(* Logix 5000 AddOnInstructionDefinition export Banner_Q90R2_KD_Param_v4; software revision 33.00 *)

TYPE Banner_IOL_Port_v4 :   // UDT that has all of the data items necessary to communicate with a specific Port on a IO-Link Master
STRUCT
   Port_Controlled : INT;   // Each bit represents a port on an IO-Link Master. Set to 1 to tell AOI to control that port.
   Port_Activate : INT;   // Each bit represents a port on an IO-Link Master. When ON that port will process any commands in queue.
   Port_Read : INT;   // Each bit represents a port on an IO-Link Master. Used to determine when device AOI has requested a Read command.
   Port_Write : INT;   // Each bit represents a port on an IO-Link Master. Used to determine when device AOI has requested a Write command.
   Port_RW_Complete : INT;   // Each bit represents a port on an IO-Link Master. Tells device AOI that Read or Write request has been completed.
   Port_Device_Read : INT;
   Data_Transfer : SINT[190];   // Array to transfer data from IO-Master to device AOIs.
END_STRUCT
END_TYPE

TYPE Banner_Q90R2KD_Config_v4 :
STRUCT
   Response_Speed : SINT;   // 0 = Fast, 1 = Medium, 2 = Slow
   Detection_Sensitivity : SINT;   // 0 = High, 1 = Standard.
   LEDs_Disabled : SINT;   // 0 = Enabled, 1 = Disabled.
   Output_Polarity : SINT;   // 0 = NPN, 1 = PNP
   Process_Data_Measurement : SINT;   // 0 = Radial, 1 = Rectangular.
   Remote_Input_Mode : SINT;   // 0 = Disabled, 1 = Teach
   Amplitude_Threshold : DINT;   // 100 to 100000. Minimum amplitude required for target detection.
   Limit_Filter_Enabled : SINT;   // 0 = Disabled, 1 = Enabled. Rate of change filter for the distance meansurement.
   Limit_Filter_Positive_Hold_Time : DINT;   // 50 to 3600000. Hold time for when distance change exceeds positive window.
   Limit_Filter_Negative_Hold_Time : DINT;   // 50 to 3600000. Hold time for when distance change exceeds negative window.
   Limit_Filter_Positive_Distance : DINT;   // 0 to 1000. Window size for distance changes going away from sensor (set 0 to disable)
   Limit_Filter_Negative_Distance : DINT;   // 0 to 1000. Window size for distance changes going towards sensor (set 0 to disable)
   Primary_Output_Mode : SINT;   // 0 = Independent Output, 1 = Complementary Output, 2 = Pulse Frequency Output.
   Secondary_Output_Mode : SINT;   // 0 = Independent Output, 1 = Complementary Output, 2 = Pulse Frequency Output.
END_STRUCT
END_TYPE

TYPE Banner_Q90R2KD_Direct_v4 :
STRUCT
   Master_Cycle_Time : INT;
   Min_Cycle_Time : INT;
   M_Sequence_Capability : INT;
   IO_Link_Version_ID : INT;
   Process_Data_Input_Length : INT;
   Process_Data_Output_Length : INT;
   Combined_Vendor_ID : DINT;   // IO-Link Vendor ID
   Vendor_ID1 : INT;
   Vendor_ID2 : INT;
   Combined_Device_ID : DINT;   // IO-Link Device ID
   Device_ID1 : INT;
   Device_ID2 : INT;
   Device_ID3 : INT;
END_STRUCT
END_TYPE

TYPE Banner_Q90R2KD_Pulse_v4 :
STRUCT
   Measurement : SINT;   // 0 = Distance or Y, 1 = Velocity. Measurement to use for PFM output.
   Frequency_SP1 : INT;   // 100 to 600. The frequency corresponding to a target at the SP1 measurement.
   Frequency_SP2 : INT;   // 100 to 600. The frequency corresponding to a target at the SP1 measurement.
   Loss_of_Signal : SINT;   // 0 = Hold, 1 = Low, 2 = High.
   Distance_SP1 : DINT;   // Distance SP1 swithc point in Switch or Window mode.
   Distance_SP2 : DINT;   // Distance SP2 switch point in Window mode only.
   Y_SP1 : DINT;   // Y SP1 switch point in Switch or Window mode.
   Y_SP2 : DINT;   // Y SP2 switch point in Window mode only.
   Velocity_SP1 : DINT;   // Velocity SP1 switch point.
   Velocity_SP2 : DINT;   // Velocity SP2 switch point.
END_STRUCT
END_TYPE

TYPE Banner_Q90R2KD_RD_v4 :   // UDT that stores the Read Data for a Q90R2KD.
STRUCT
   Direct : Banner_Q90R2KD_Direct_v4;   // Direct Parameters.
   Serial_Number : STRING;
   Teach_Status : Banner_Q90R2KD_Teach_Status_v4;
   Status : Banner_Q90R2KD_Status_v4;
   All_Time_Run_Time : DINT;   // Read only counter that tracks the total time sensor has been running since manufacture. Value in Hours.
END_STRUCT
END_TYPE

TYPE Banner_Q90R2KD_SSC_v4 :
STRUCT
   Distance_SP1 : DINT;   // SP1 switch point in Switch or Window mode.
   Distance_SP2 : DINT;   // SP2 switch point in Window mode only.
   Distance_Hysteresis : INT;
   Y_SP1 : DINT;   // Y SP1 siwtch point in Switch or Window mode.
   Y_SP2 : DINT;   // Y SP2 switch point in Window mode only.
   Y_Hysteresis : DINT;
   Switch_Point_Logic : INT;   // 0 = Light Operate - Output is On while target is detected, 1 = Dark Operate - Output is Off while target is detected.
   Distance_Y_Setpoint_Mode : INT;   // 1 = Switch Mode/Single Point Mode, 2 = Window Mode.
   Delay_On : DINT;   // 0 to 60000.
   Delay_Off : DINT;   // 0 to 60000.
   Distance_Window_Size : DINT;   // This will set the size of the distance window after a teach. Window size will be +/- xmm where x is the value written.
   Distance_User_Teach_Offset : DINT;   // Distance offset applied to taught switch point.
   Beam_Angle_Window_Size : DINT;   // This will set the size of the beam angle window after a teach. Window size will be +/- xmm where x is the value written.
   Beam_Angle_User_Teach_Offset : DINT;   // Beam Angle offset applied to taught switch point.
   X_Window_Size : DINT;   // This will set the size of the X window after a teach. Window size will be +/- xmm where x is the value written.
   X_User_Teach_Offset : DINT;   // X offset applied to taught switch point.
   Y_Window_Size : DINT;   // This will set the size of the Y window after a teach. Window size will be +/- xmm where x is the value written.
   Y_User_Teach_Offset : DINT;   // Y offset applied to taught switch point.
   Peak_Select_Mode : SINT;   // 0 = First Peak, 1 = Strongest Peak.
   Beam_Angle_SP1 : INT;   // Beam Angle SP1 Switch point.
   Beam_Angle_SP2 : INT;   // Beam Angle SP2 switch point.
   Beam_Angle_Hysteresis : SINT;   // Hysteresis value for the beam angle switchpoint.
   X_SP1 : DINT;   // X SP1 switch point.
   X_SP2 : DINT;   // X SP2 switch point.
   X_Hysteresis : INT;   // Hysteresis value for the X switchpoint.
END_STRUCT
END_TYPE

TYPE Banner_Q90R2KD_Status_v4 :
STRUCT
   SSC1_State : SINT;   // 0 = Inactive, 1 = Active.
   SSC1_Stability : SINT;   // 0 = No target, 1 = Marginal target, 2 = Strong target.
   SSC1_Distance_or_X : DINT;
   SSC1_Beam_Angle_or_Y : DINT;
   SSC1_Velocity : DINT;
   SSC1_Signal_Strength : SINT;
   SSC2_State : SINT;   // 0 = Inactive, 1 = Active.
   SSC2_Stability : SINT;   // 0 = No target, 1 = Marginal target, 2 = Strong target.
   SSC2_Distance_or_X : DINT;
   SSC2_Beam_Angle_or_Y : DINT;
   SSC2_Velocity : DINT;
   SSC2_Signal_Strength : SINT;
   Fault_Status : SINT;   // 0 = No fault present, 1 = Fault present.
   Temperature : DINT;
   Last_Temperature : DINT;
END_STRUCT
END_TYPE

TYPE Banner_Q90R2KD_Target_Filters_v4 :
STRUCT
   Detection_Area : SINT;   // 0 = Radial, 1 = Rectangular.
   Min_Active_Sensing_Distance : DINT;   // Near radial distance measurement limit of sensing range.
   Max_Active_Sensing_Distance : DINT;   // Far radial distance measurement limit of sensing range.
   Min_Active_Sensing_Y : DINT;   // Near Y coordinate measurement limit of sensing range.
   Max_Active_Sensing_Y : DINT;   // Far Y coordinate measurment limit of sensing range.
   Velocity_Filter : INT;   // 0 = All Target Velocities, 1 = Dynamix Targets Only, 2 = Approaching Targets Only, 3 = Receding Targets Only, 4 = Custom.
   Min_Velocity : DINT;   // Minimum velocity limit of sensing range.
   Max_Velocity : DINT;   // Maximum velocity lmiit of sensing range.
   Velocity_Hysteresis : DINT;   // Hysteresis value for the velocity switchpoint.
END_STRUCT
END_TYPE

TYPE Banner_Q90R2KD_Teach_Status_v4 :
STRUCT
   Teach_State : SINT;   // 0 = Idle, 1 = SP1 Success, 2 = SP2 Success, 3 = SP1 SP2 Success, 4 = Wait for command, 5 = Busy, 7 = Error
   SP1_TP1 : SINT;
   SP1_TP2 : SINT;
   SP2_TP1 : SINT;
   SP2_TP2 : SINT;
END_STRUCT
END_TYPE

TYPE Banner_Q90R2KD_v4 :   // All of the parameters for a Q90R2KD.
STRUCT
   Initial_Global_Read : BOOL;   // Determines if all of the IO-Link data has been read into the PLC yet
   Command : INT;   // Value placed in here will activate a read or write to a specifc IO-Link Index
   Read : Banner_Q90R2KD_RD_v4;   // Read Only Data
   Write : Banner_Q90R2KD_WD_v4;   // Write Data
   Reset : BOOL;   // Resets AOI. This will force a complete parameter read of the sensor.
END_STRUCT
END_TYPE

TYPE Banner_Q90R2KD_WD_v4 :   // UDT that stores the Write Data for a Q90R2KD.
STRUCT
   System_Command : INT;   // See IODD file for list of commands that can be activated via the System Command interface
   Teach_in_Channel : SINT;   // 0 = Default, 1 = BDC1, 2 = BDC2
   SSC1 : Banner_Q90R2KD_SSC_v4;
   SSC2 : Banner_Q90R2KD_SSC_v4;
   Config : Banner_Q90R2KD_Config_v4;
   Resettable_Run_Time : DINT;
   All_Time_Run_Time_Event_Time : DINT;
   Resettable_Run_Time_Event_Time : DINT;
   Target_Filters : Banner_Q90R2KD_Target_Filters_v4;
   Pulse1 : Banner_Q90R2KD_Pulse_v4;
   Pulse2 : Banner_Q90R2KD_Pulse_v4;
END_STRUCT
END_TYPE

ADD_ON_INSTRUCTION Banner_Q90R2_KD_Param_v4   (* revision 4.0, vendor Banner Engineering *)
// AOI to read and write parameter data to an IO-Link Q90R2 Dual Discrete.
VAR_IN_OUT
   Q90R2KD : Banner_Q90R2KD_v4; {required}
   Port_Data : Banner_IOL_Port_v4; {required}
END_VAR
VAR_INPUT
   Port : DINT; {required}
END_VAR
VAR
   Local_Control : DINT; {access None}
   Global_Read_Command_Value : INT; {access None}
   Global_Write_Command_Value : INT; {access None}
   Command_Being_Processed : BOOL; {access None}
   Update_Archive : BOOL; {access None}
   Index_Write_Inprocess : DINT; {access None}
   Index_Write_Control : DINT; {access None}
   Inprocess_Index : DINT; {access None}
END_VAR

ROUTINE Logic   (* ladder *)
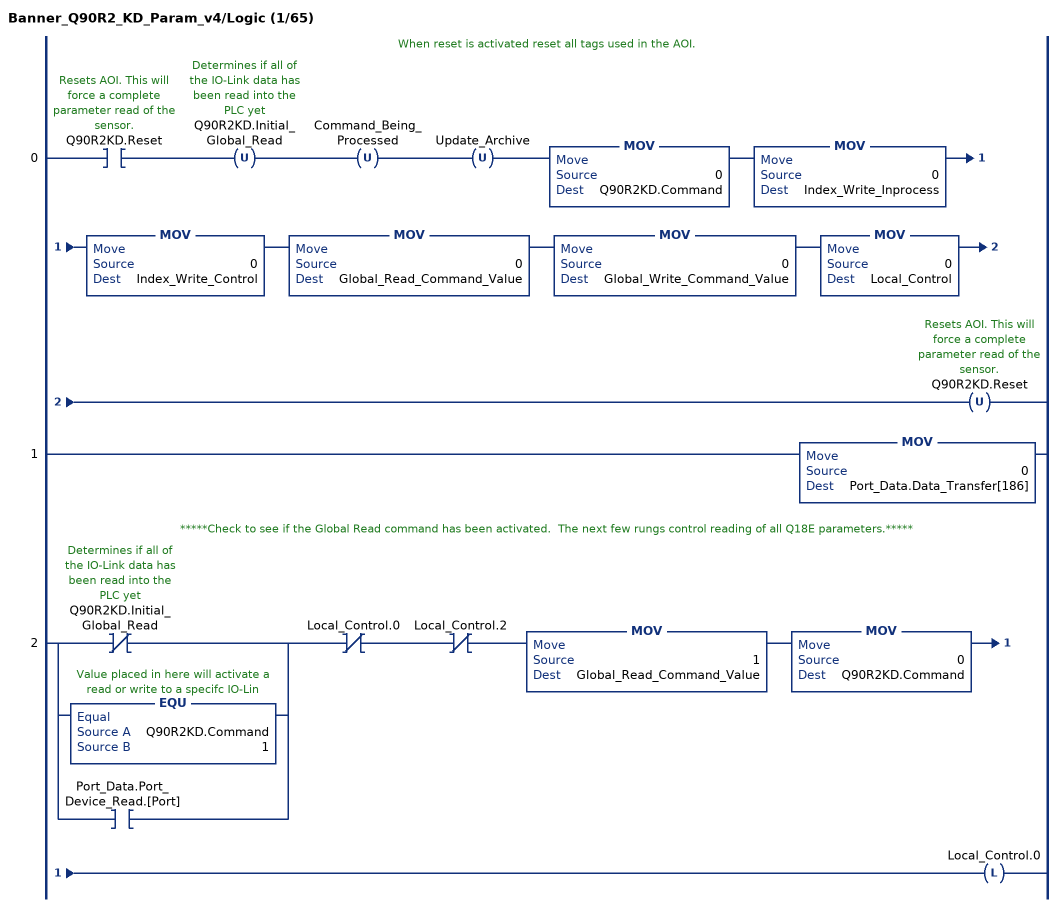
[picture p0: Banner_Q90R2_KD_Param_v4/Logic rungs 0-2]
   // When reset is activated reset all tags used in the AOI.
   0: XIC(Q90R2KD.Reset)OTU(Q90R2KD.Initial_Global_Read)OTU(Command_Being_Processed)OTU(Update_Archive)MOV(0,Q90R2KD.Command)MOV(0,Index_Write_Inprocess)MOV(0,Index_Write_Control)MOV(0,Global_Read_Command_Value)MOV(0,Global_Write_Command_Value)MOV(0,Local_Control)OTU(Q90R2KD.Reset);
   1: MOV(0,Port_Data.Data_Transfer[186]);
   // *****Check to see if the Global Read command has been activated.  The next few rungs control reading of all Q18E parameters.*****
   2: [XIO(Q90R2KD.Initial_Global_Read) ,EQU(Q90R2KD.Command,1) ,XIC(Port_Data.Port_Device_Read.[Port]) ]XIO(Local_Control.0)XIO(Local_Control.2)MOV(1,Global_Read_Command_Value)MOV(0,Q90R2KD.Command)OTL(Local_Control.0);
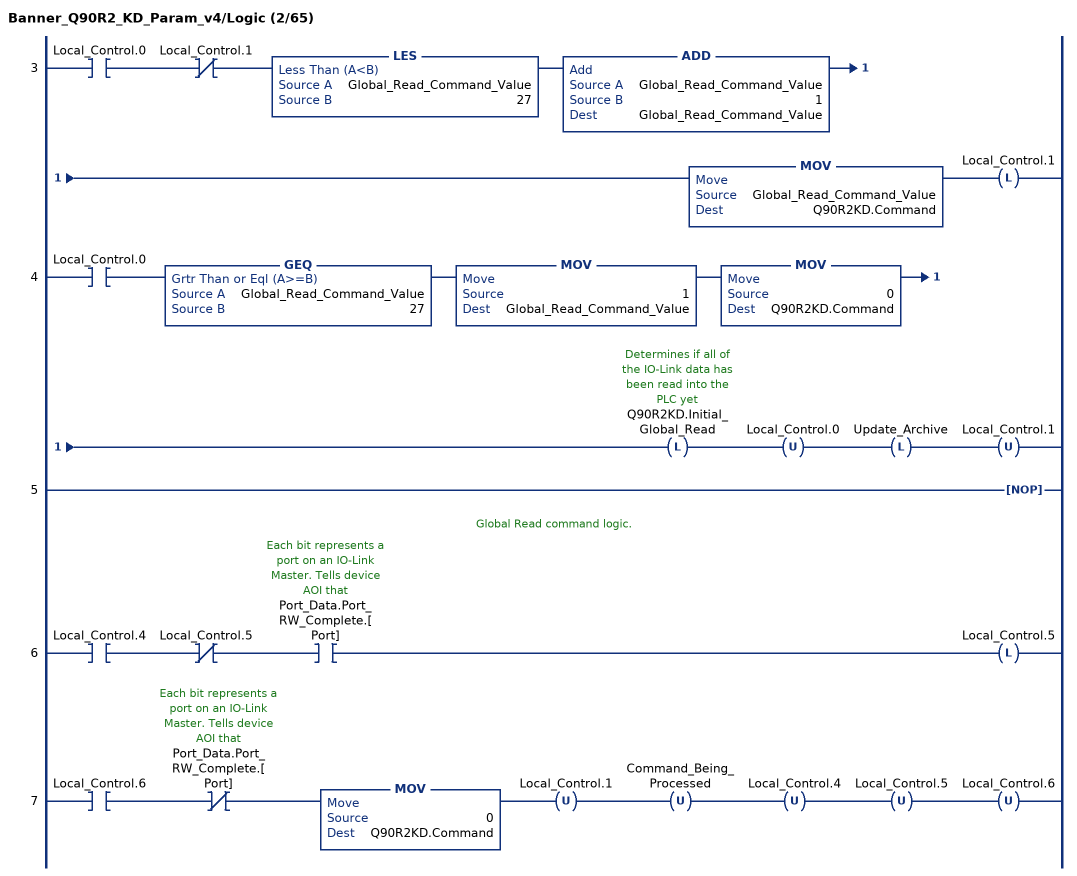
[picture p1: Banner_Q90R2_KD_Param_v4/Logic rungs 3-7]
   3: XIC(Local_Control.0)XIO(Local_Control.1)LES(Global_Read_Command_Value,27)ADD(Global_Read_Command_Value,1,Global_Read_Command_Value)MOV(Global_Read_Command_Value,Q90R2KD.Command)OTL(Local_Control.1);
   4: XIC(Local_Control.0)GEQ(Global_Read_Command_Value,27)MOV(1,Global_Read_Command_Value)MOV(0,Q90R2KD.Command)OTL(Q90R2KD.Initial_Global_Read)OTU(Local_Control.0)OTL(Update_Archive)OTU(Local_Control.1);
   5: NOP();
   // Global Read command logic.
   6: XIC(Local_Control.4)XIO(Local_Control.5)XIC(Port_Data.Port_RW_Complete.[Port])OTL(Local_Control.5);
   7: XIC(Local_Control.6)XIO(Port_Data.Port_RW_Complete.[Port])MOV(0,Q90R2KD.Command)OTU(Local_Control.1)OTU(Command_Being_Processed)OTU(Local_Control.4)OTU(Local_Control.5)OTU(Local_Control.6);
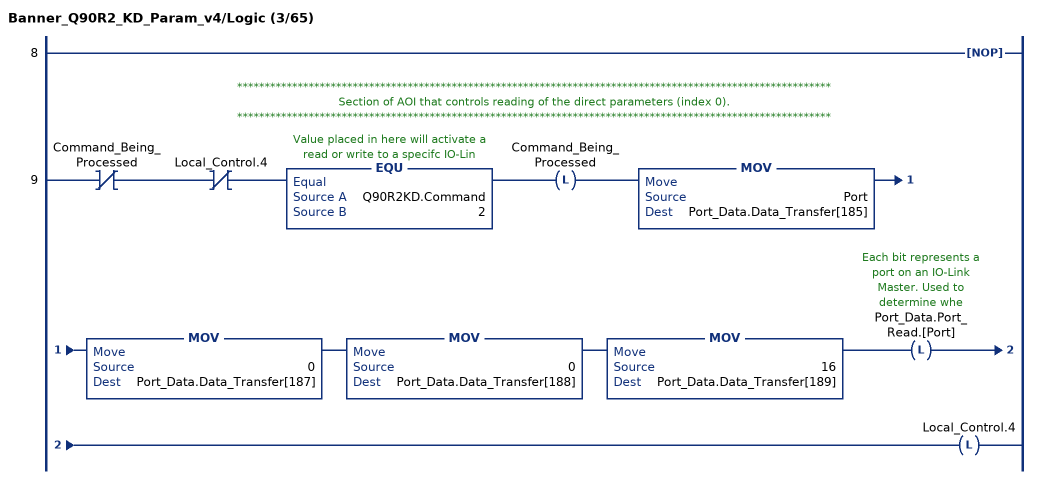
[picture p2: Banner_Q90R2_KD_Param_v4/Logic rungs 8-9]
   8: NOP();
   // ************************************************************************************************************
   // Section of AOI that controls reading of the direct parameters (index 0).
   // ************************************************************************************************************
   9: XIO(Command_Being_Processed)XIO(Local_Control.4)EQU(Q90R2KD.Command,2)OTL(Command_Being_Processed)MOV(Port,Port_Data.Data_Transfer[185])MOV(0,Port_Data.Data_Transfer[187])MOV(0,Port_Data.Data_Transfer[188])MOV(16,Port_Data.Data_Transfer[189])OTL(Port_Data.Port_Read.[Port])OTL(Local_Control.4);
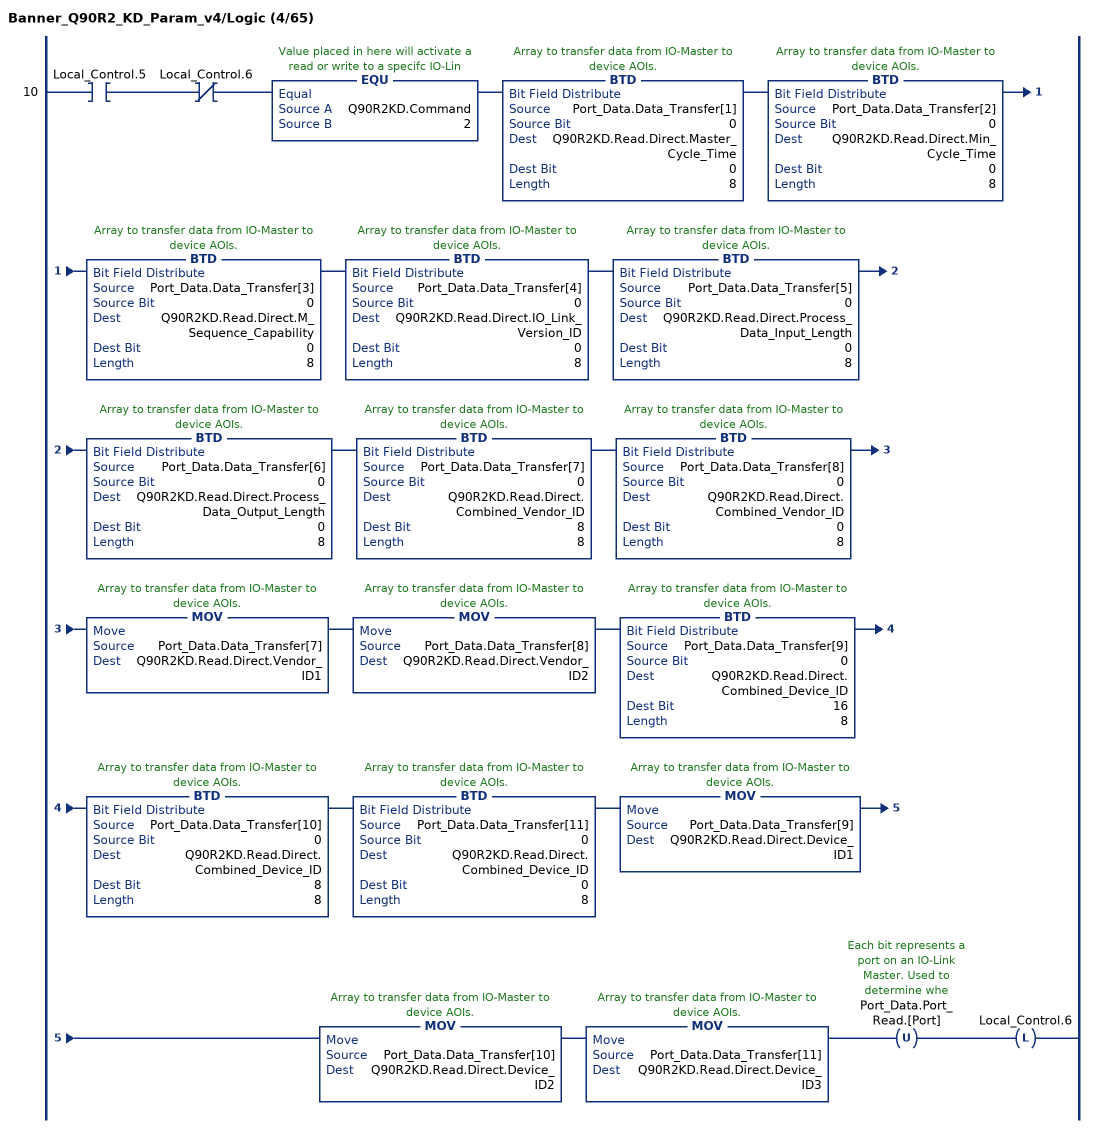
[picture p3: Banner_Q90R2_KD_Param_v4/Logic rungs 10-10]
   10: XIC(Local_Control.5)XIO(Local_Control.6)EQU(Q90R2KD.Command,2)BTD(Port_Data.Data_Transfer[1],0,Q90R2KD.Read.Direct.Master_Cycle_Time,0,8)BTD(Port_Data.Data_Transfer[2],0,Q90R2KD.Read.Direct.Min_Cycle_Time,0,8)BTD(Port_Data.Data_Transfer[3],0,Q90R2KD.Read.Direct.M_Sequence_Capability,0,8)BTD(Port_Data.Data_Transfer[4],0,Q90R2KD.Read.Direct.IO_Link_Version_ID,0,8)BTD(Port_Data.Data_Transfer[5],0,Q90R2KD.Read.Direct.Process_Data_Input_Length,0,8)BTD(Port_Data.Data_Transfer[6],0,Q90R2KD.Read.Direct.Process_Data_Output_Length,0,8)BTD(Port_Data.Data_Transfer[7],0,Q90R2KD.Read.Direct.Combined_Vendor_ID,8,8)BTD(Port_Data.Data_Transfer[8],0,Q90R2KD.Read.Direct.Combined_Vendor_ID,0,8)MOV(Port_Data.Data_Transfer[7],Q90R2KD.Read.Direct.Vendor_ID1)MOV(Port_Data.Data_Transfer[8],Q90R2KD.Read.Direct.Vendor_ID2)BTD(Port_Data.Data_Transfer[9],0,Q90R2KD.Read.Direct.Combined_Device_ID,16,8)BTD(Port_Data.Data_Transfer[10],0,Q90R2KD.Read.Direct.Combined_Device_ID,8,8)BTD(Port_Data.Data_Transfer[11],0,Q90R2KD.Read.Direct.Combined_Device_ID,0,8)MOV(Port_Data.Data_Transfer[9],Q90R2KD.Read.Direct.Device_ID1)MOV(Port_Data.Data_Transfer[10],Q90R2KD.Read.Direct.Device_ID2)MOV(Port_Data.Data_Transfer[11],Q90R2KD.Read.Direct.Device_ID3)OTU(Port_Data.Port_Read.[Port])OTL(Local_Control.6);
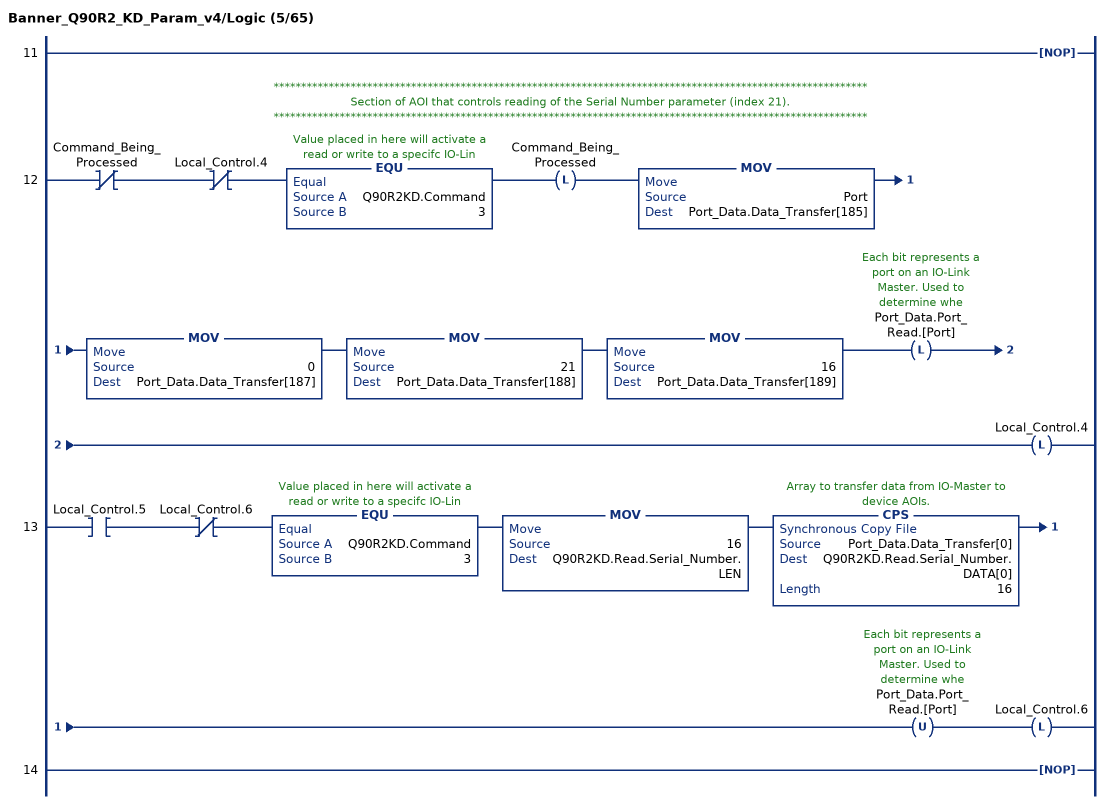
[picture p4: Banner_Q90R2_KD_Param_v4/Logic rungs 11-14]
   11: NOP();
   // ************************************************************************************************************
   // Section of AOI that controls reading of the Serial Number parameter (index 21).
   // ************************************************************************************************************
   12: XIO(Command_Being_Processed)XIO(Local_Control.4)EQU(Q90R2KD.Command,3)OTL(Command_Being_Processed)MOV(Port,Port_Data.Data_Transfer[185])MOV(0,Port_Data.Data_Transfer[187])MOV(21,Port_Data.Data_Transfer[188])MOV(16,Port_Data.Data_Transfer[189])OTL(Port_Data.Port_Read.[Port])OTL(Local_Control.4);
   13: XIC(Local_Control.5)XIO(Local_Control.6)EQU(Q90R2KD.Command,3)MOV(16,Q90R2KD.Read.Serial_Number.LEN)CPS(Port_Data.Data_Transfer[0],Q90R2KD.Read.Serial_Number.DATA[0],16)OTU(Port_Data.Port_Read.[Port])OTL(Local_Control.6);
   14: NOP();
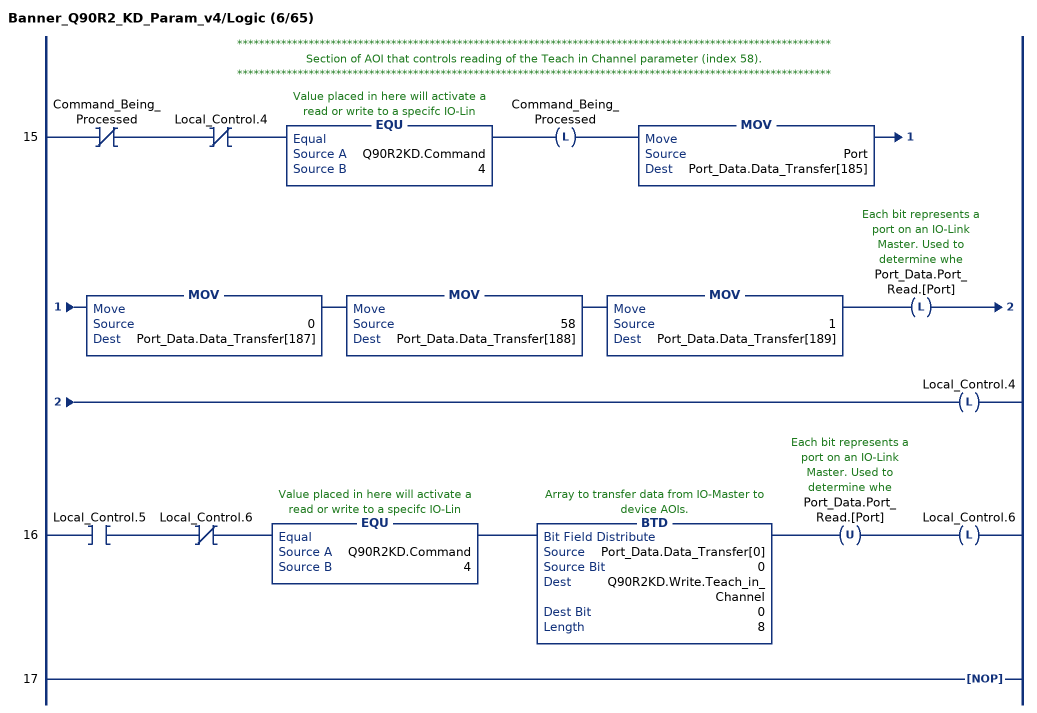
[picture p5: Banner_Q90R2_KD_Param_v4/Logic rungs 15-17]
   // ************************************************************************************************************
   // Section of AOI that controls reading of the Teach in Channel parameter (index 58).
   // ************************************************************************************************************
   15: XIO(Command_Being_Processed)XIO(Local_Control.4)EQU(Q90R2KD.Command,4)OTL(Command_Being_Processed)MOV(Port,Port_Data.Data_Transfer[185])MOV(0,Port_Data.Data_Transfer[187])MOV(58,Port_Data.Data_Transfer[188])MOV(1,Port_Data.Data_Transfer[189])OTL(Port_Data.Port_Read.[Port])OTL(Local_Control.4);
   16: XIC(Local_Control.5)XIO(Local_Control.6)EQU(Q90R2KD.Command,4)BTD(Port_Data.Data_Transfer[0],0,Q90R2KD.Write.Teach_in_Channel,0,8)OTU(Port_Data.Port_Read.[Port])OTL(Local_Control.6);
   17: NOP();
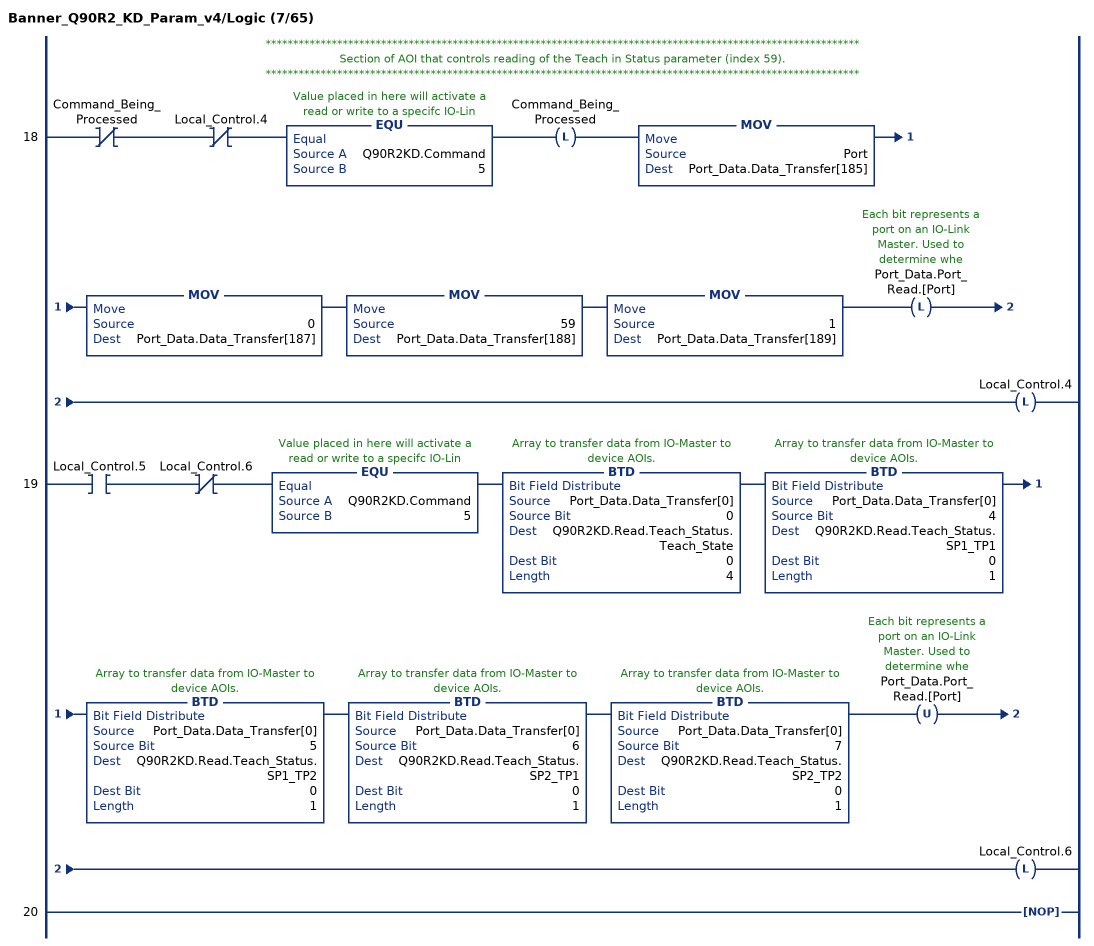
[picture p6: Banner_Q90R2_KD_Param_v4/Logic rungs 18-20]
   // ************************************************************************************************************
   // Section of AOI that controls reading of the Teach in Status parameter (index 59).
   // ************************************************************************************************************
   18: XIO(Command_Being_Processed)XIO(Local_Control.4)EQU(Q90R2KD.Command,5)OTL(Command_Being_Processed)MOV(Port,Port_Data.Data_Transfer[185])MOV(0,Port_Data.Data_Transfer[187])MOV(59,Port_Data.Data_Transfer[188])MOV(1,Port_Data.Data_Transfer[189])OTL(Port_Data.Port_Read.[Port])OTL(Local_Control.4);
   19: XIC(Local_Control.5)XIO(Local_Control.6)EQU(Q90R2KD.Command,5)BTD(Port_Data.Data_Transfer[0],0,Q90R2KD.Read.Teach_Status.Teach_State,0,4)BTD(Port_Data.Data_Transfer[0],4,Q90R2KD.Read.Teach_Status.SP1_TP1,0,1)BTD(Port_Data.Data_Transfer[0],5,Q90R2KD.Read.Teach_Status.SP1_TP2,0,1)BTD(Port_Data.Data_Transfer[0],6,Q90R2KD.Read.Teach_Status.SP2_TP1,0,1)BTD(Port_Data.Data_Transfer[0],7,Q90R2KD.Read.Teach_Status.SP2_TP2,0,1)OTU(Port_Data.Port_Read.[Port])OTL(Local_Control.6);
   20: NOP();
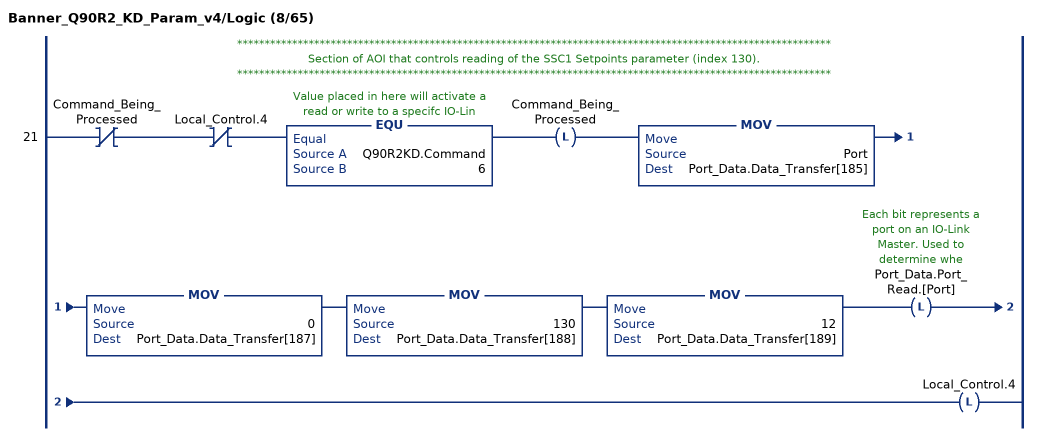
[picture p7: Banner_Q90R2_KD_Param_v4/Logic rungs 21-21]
   // ************************************************************************************************************
   // Section of AOI that controls reading of the SSC1 Setpoints parameter (index 130).
   // ************************************************************************************************************
   21: XIO(Command_Being_Processed)XIO(Local_Control.4)EQU(Q90R2KD.Command,6)OTL(Command_Being_Processed)MOV(Port,Port_Data.Data_Transfer[185])MOV(0,Port_Data.Data_Transfer[187])MOV(130,Port_Data.Data_Transfer[188])MOV(12,Port_Data.Data_Transfer[189])OTL(Port_Data.Port_Read.[Port])OTL(Local_Control.4);
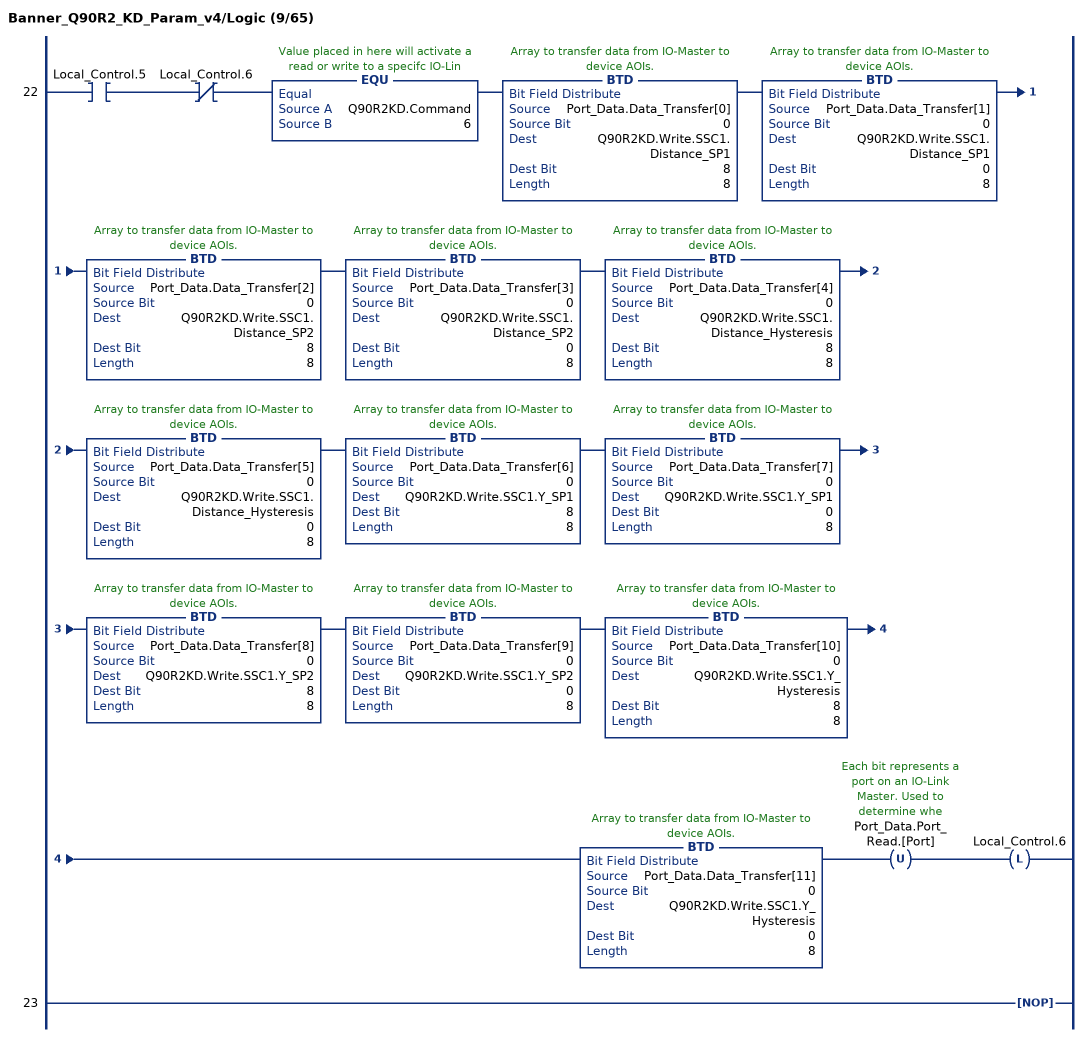
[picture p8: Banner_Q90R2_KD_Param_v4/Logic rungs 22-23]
   22: XIC(Local_Control.5)XIO(Local_Control.6)EQU(Q90R2KD.Command,6)BTD(Port_Data.Data_Transfer[0],0,Q90R2KD.Write.SSC1.Distance_SP1,8,8)BTD(Port_Data.Data_Transfer[1],0,Q90R2KD.Write.SSC1.Distance_SP1,0,8)BTD(Port_Data.Data_Transfer[2],0,Q90R2KD.Write.SSC1.Distance_SP2,8,8)BTD(Port_Data.Data_Transfer[3],0,Q90R2KD.Write.SSC1.Distance_SP2,0,8)BTD(Port_Data.Data_Transfer[4],0,Q90R2KD.Write.SSC1.Distance_Hysteresis,8,8)BTD(Port_Data.Data_Transfer[5],0,Q90R2KD.Write.SSC1.Distance_Hysteresis,0,8)BTD(Port_Data.Data_Transfer[6],0,Q90R2KD.Write.SSC1.Y_SP1,8,8)BTD(Port_Data.Data_Transfer[7],0,Q90R2KD.Write.SSC1.Y_SP1,0,8)BTD(Port_Data.Data_Transfer[8],0,Q90R2KD.Write.SSC1.Y_SP2,8,8)BTD(Port_Data.Data_Transfer[9],0,Q90R2KD.Write.SSC1.Y_SP2,0,8)BTD(Port_Data.Data_Transfer[10],0,Q90R2KD.Write.SSC1.Y_Hysteresis,8,8)BTD(Port_Data.Data_Transfer[11],0,Q90R2KD.Write.SSC1.Y_Hysteresis,0,8)OTU(Port_Data.Port_Read.[Port])OTL(Local_Control.6);
   23: NOP();
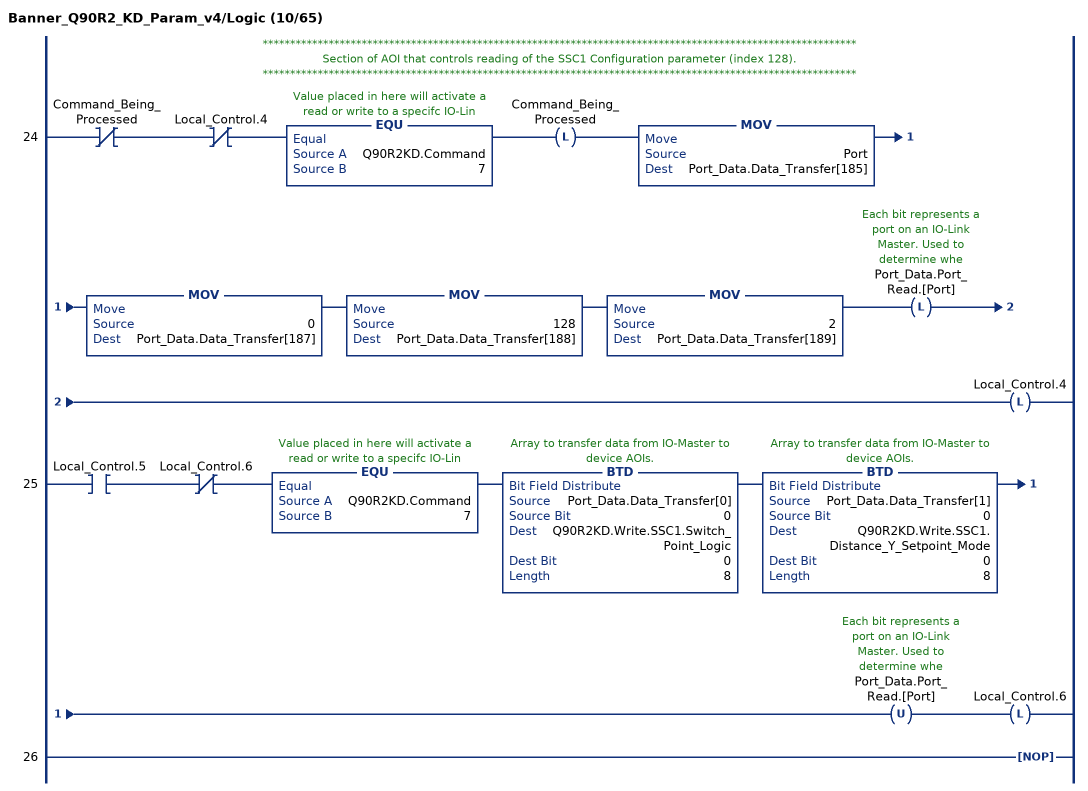
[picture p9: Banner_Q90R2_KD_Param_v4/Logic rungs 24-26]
   // ************************************************************************************************************
   // Section of AOI that controls reading of the SSC1 Configuration parameter (index 128).
   // ************************************************************************************************************
   24: XIO(Command_Being_Processed)XIO(Local_Control.4)EQU(Q90R2KD.Command,7)OTL(Command_Being_Processed)MOV(Port,Port_Data.Data_Transfer[185])MOV(0,Port_Data.Data_Transfer[187])MOV(128,Port_Data.Data_Transfer[188])MOV(2,Port_Data.Data_Transfer[189])OTL(Port_Data.Port_Read.[Port])OTL(Local_Control.4);
   25: XIC(Local_Control.5)XIO(Local_Control.6)EQU(Q90R2KD.Command,7)BTD(Port_Data.Data_Transfer[0],0,Q90R2KD.Write.SSC1.Switch_Point_Logic,0,8)BTD(Port_Data.Data_Transfer[1],0,Q90R2KD.Write.SSC1.Distance_Y_Setpoint_Mode,0,8)OTU(Port_Data.Port_Read.[Port])OTL(Local_Control.6);
   26: NOP();
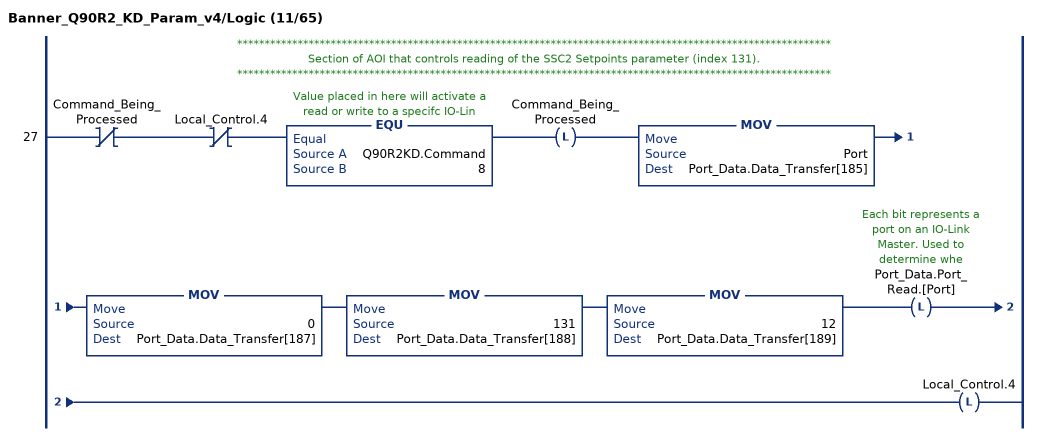
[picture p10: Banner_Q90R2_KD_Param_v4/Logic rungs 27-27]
   // ************************************************************************************************************
   // Section of AOI that controls reading of the SSC2 Setpoints parameter (index 131).
   // ************************************************************************************************************
   27: XIO(Command_Being_Processed)XIO(Local_Control.4)EQU(Q90R2KD.Command,8)OTL(Command_Being_Processed)MOV(Port,Port_Data.Data_Transfer[185])MOV(0,Port_Data.Data_Transfer[187])MOV(131,Port_Data.Data_Transfer[188])MOV(12,Port_Data.Data_Transfer[189])OTL(Port_Data.Port_Read.[Port])OTL(Local_Control.4);
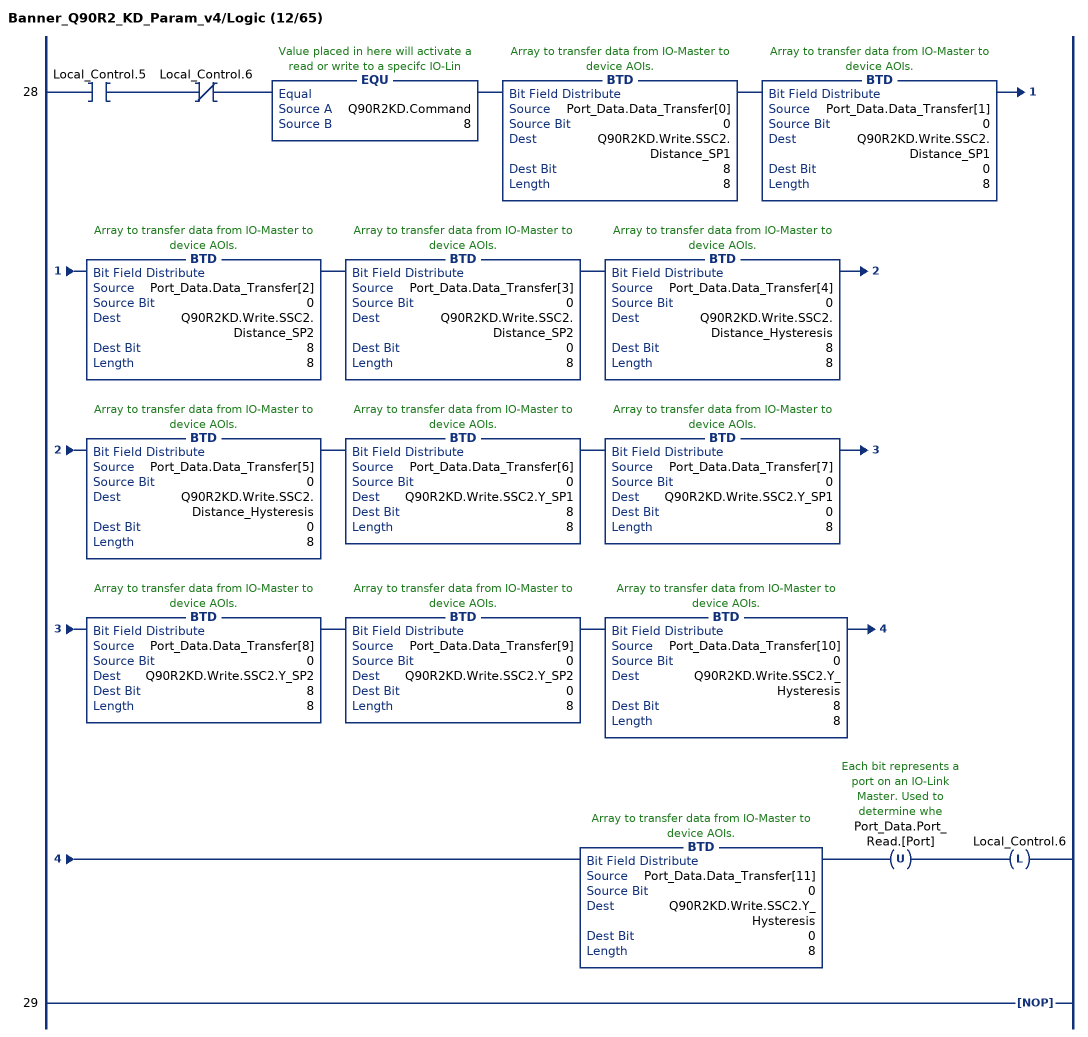
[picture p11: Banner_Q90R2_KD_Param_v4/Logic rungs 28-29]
   28: XIC(Local_Control.5)XIO(Local_Control.6)EQU(Q90R2KD.Command,8)BTD(Port_Data.Data_Transfer[0],0,Q90R2KD.Write.SSC2.Distance_SP1,8,8)BTD(Port_Data.Data_Transfer[1],0,Q90R2KD.Write.SSC2.Distance_SP1,0,8)BTD(Port_Data.Data_Transfer[2],0,Q90R2KD.Write.SSC2.Distance_SP2,8,8)BTD(Port_Data.Data_Transfer[3],0,Q90R2KD.Write.SSC2.Distance_SP2,0,8)BTD(Port_Data.Data_Transfer[4],0,Q90R2KD.Write.SSC2.Distance_Hysteresis,8,8)BTD(Port_Data.Data_Transfer[5],0,Q90R2KD.Write.SSC2.Distance_Hysteresis,0,8)BTD(Port_Data.Data_Transfer[6],0,Q90R2KD.Write.SSC2.Y_SP1,8,8)BTD(Port_Data.Data_Transfer[7],0,Q90R2KD.Write.SSC2.Y_SP1,0,8)BTD(Port_Data.Data_Transfer[8],0,Q90R2KD.Write.SSC2.Y_SP2,8,8)BTD(Port_Data.Data_Transfer[9],0,Q90R2KD.Write.SSC2.Y_SP2,0,8)BTD(Port_Data.Data_Transfer[10],0,Q90R2KD.Write.SSC2.Y_Hysteresis,8,8)BTD(Port_Data.Data_Transfer[11],0,Q90R2KD.Write.SSC2.Y_Hysteresis,0,8)OTU(Port_Data.Port_Read.[Port])OTL(Local_Control.6);
   29: NOP();
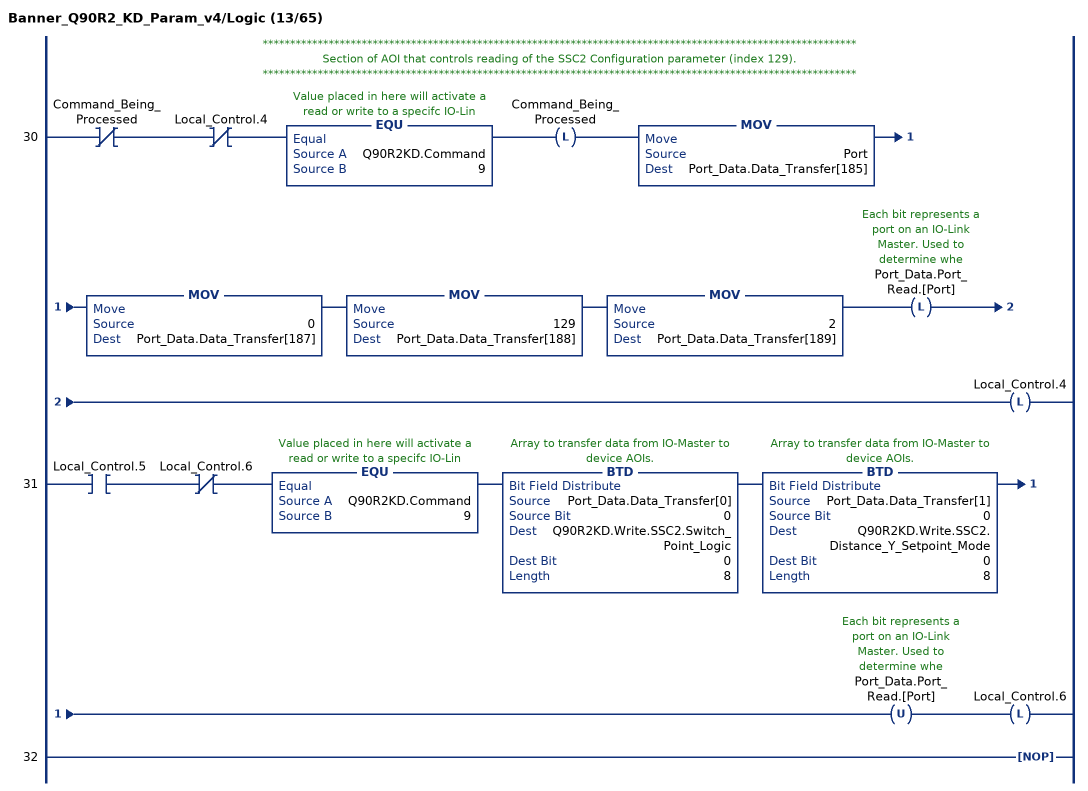
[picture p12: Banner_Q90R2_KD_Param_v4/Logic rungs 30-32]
   // ************************************************************************************************************
   // Section of AOI that controls reading of the SSC2 Configuration parameter (index 129).
   // ************************************************************************************************************
   30: XIO(Command_Being_Processed)XIO(Local_Control.4)EQU(Q90R2KD.Command,9)OTL(Command_Being_Processed)MOV(Port,Port_Data.Data_Transfer[185])MOV(0,Port_Data.Data_Transfer[187])MOV(129,Port_Data.Data_Transfer[188])MOV(2,Port_Data.Data_Transfer[189])OTL(Port_Data.Port_Read.[Port])OTL(Local_Control.4);
   31: XIC(Local_Control.5)XIO(Local_Control.6)EQU(Q90R2KD.Command,9)BTD(Port_Data.Data_Transfer[0],0,Q90R2KD.Write.SSC2.Switch_Point_Logic,0,8)BTD(Port_Data.Data_Transfer[1],0,Q90R2KD.Write.SSC2.Distance_Y_Setpoint_Mode,0,8)OTU(Port_Data.Port_Read.[Port])OTL(Local_Control.6);
   32: NOP();
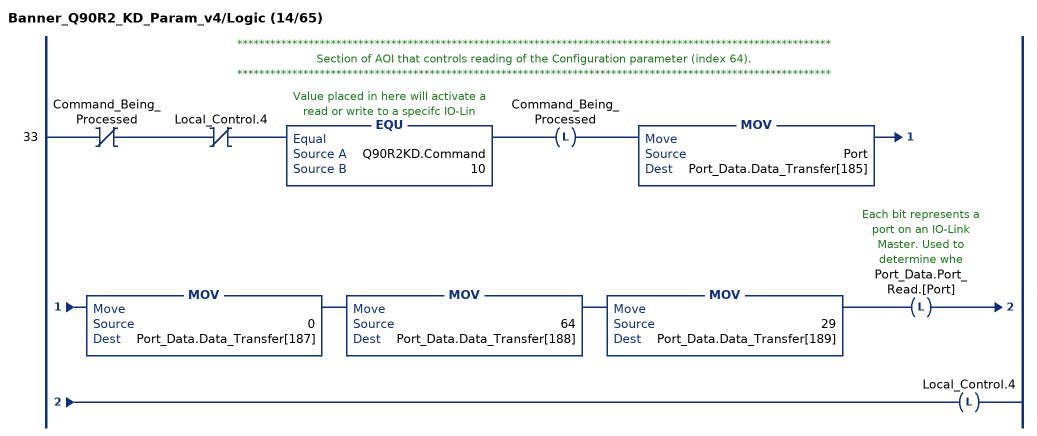
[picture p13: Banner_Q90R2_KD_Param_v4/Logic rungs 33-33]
   // ************************************************************************************************************
   // Section of AOI that controls reading of the Configuration parameter (index 64).
   // ************************************************************************************************************
   33: XIO(Command_Being_Processed)XIO(Local_Control.4)EQU(Q90R2KD.Command,10)OTL(Command_Being_Processed)MOV(Port,Port_Data.Data_Transfer[185])MOV(0,Port_Data.Data_Transfer[187])MOV(64,Port_Data.Data_Transfer[188])MOV(29,Port_Data.Data_Transfer[189])OTL(Port_Data.Port_Read.[Port])OTL(Local_Control.4);
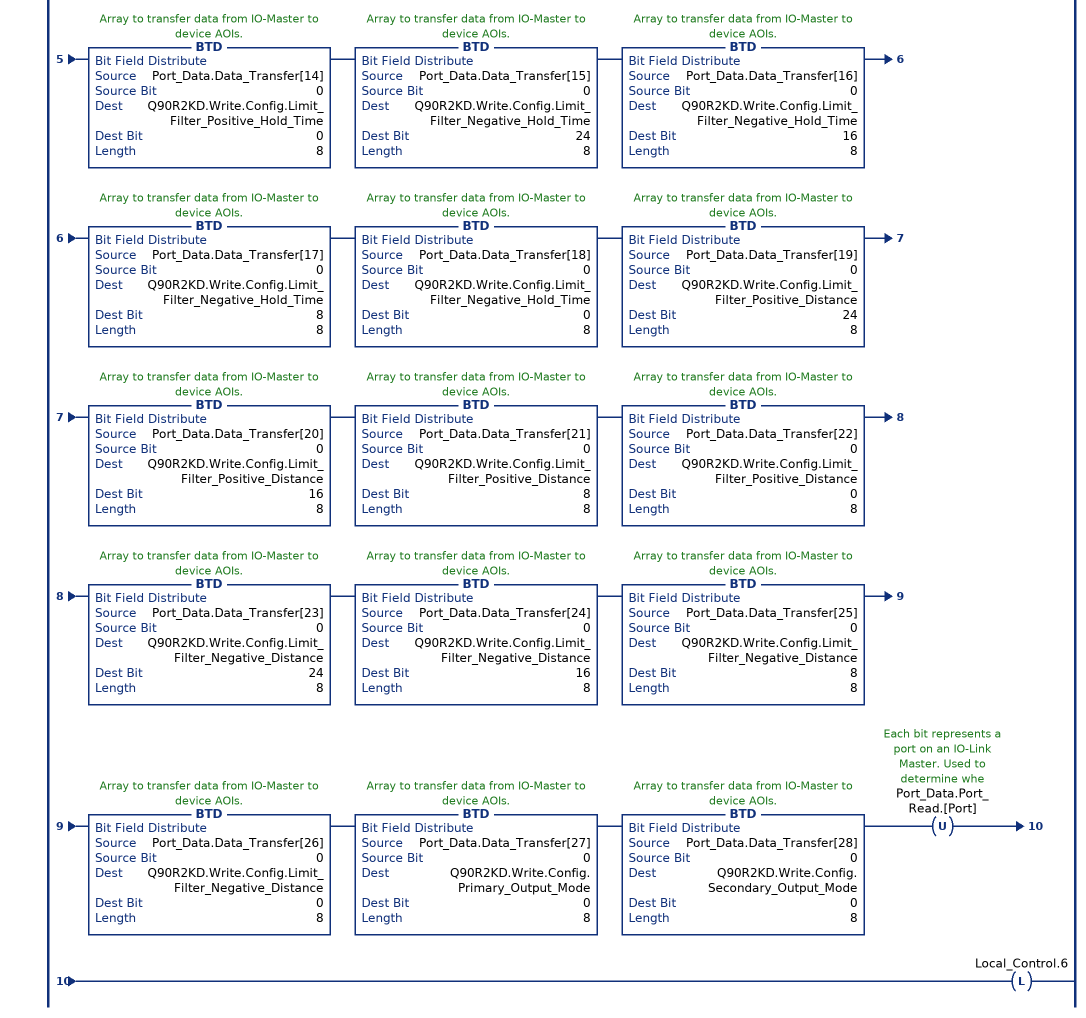
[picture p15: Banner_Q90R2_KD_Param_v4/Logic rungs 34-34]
   34: XIC(Local_Control.5)XIO(Local_Control.6)EQU(Q90R2KD.Command,10)BTD(Port_Data.Data_Transfer[0],0,Q90R2KD.Write.Config.Response_Speed,0,8)BTD(Port_Data.Data_Transfer[1],0,Q90R2KD.Write.Config.Detection_Sensitivity,0,8)BTD(Port_Data.Data_Transfer[2],0,Q90R2KD.Write.Config.LEDs_Disabled,0,8)BTD(Port_Data.Data_Transfer[3],0,Q90R2KD.Write.Config.Output_Polarity,0,8)BTD(Port_Data.Data_Transfer[4],0,Q90R2KD.Write.Config.Process_Data_Measurement,0,8)BTD(Port_Data.Data_Transfer[5],0,Q90R2KD.Write.Config.Remote_Input_Mode,0,8)BTD(Port_Data.Data_Transfer[6],0,Q90R2KD.Write.Config.Amplitude_Threshold,24,8)BTD(Port_Data.Data_Transfer[7],0,Q90R2KD.Write.Config.Amplitude_Threshold,16,8)BTD(Port_Data.Data_Transfer[8],0,Q90R2KD.Write.Config.Amplitude_Threshold,8,8)BTD(Port_Data.Data_Transfer[9],0,Q90R2KD.Write.Config.Amplitude_Threshold,0,8)BTD(Port_Data.Data_Transfer[10],0,Q90R2KD.Write.Config.Limit_Filter_Enabled,0,8)BTD(Port_Data.Data_Transfer[11],0,Q90R2KD.Write.Config.Limit_Filter_Positive_Hold_Time,24,8)BTD(Port_Data.Data_Transfer[12],0,Q90R2KD.Write.Config.Limit_Filter_Positive_Hold_Time,16,8)BTD(Port_Data.Data_Transfer[13],0,Q90R2KD.Write.Config.Limit_Filter_Positive_Hold_Time,8,8)BTD(Port_Data.Data_Transfer[14],0,Q90R2KD.Write.Config.Limit_Filter_Positive_Hold_Time,0,8)BTD(Port_Data.Data_Transfer[15],0,Q90R2KD.Write.Config.Limit_Filter_Negative_Hold_Time,24,8)BTD(Port_Data.Data_Transfer[16],0,Q90R2KD.Write.Config.Limit_Filter_Negative_Hold_Time,16,8)BTD(Port_Data.Data_Transfer[17],0,Q90R2KD.Write.Config.Limit_Filter_Negative_Hold_Time,8,8)BTD(Port_Data.Data_Transfer[18],0,Q90R2KD.Write.Config.Limit_Filter_Negative_Hold_Time,0,8)BTD(Port_Data.Data_Transfer[19],0,Q90R2KD.Write.Config.Limit_Filter_Positive_Distance,24,8)BTD(Port_Data.Data_Transfer[20],0,Q90R2KD.Write.Config.Limit_Filter_Positive_Distance,16,8)BTD(Port_Data.Data_Transfer[21],0,Q90R2KD.Write.Config.Limit_Filter_Positive_Distance,8,8)BTD(Port_Data.Data_Transfer[22],0,Q90R2KD.Write.Config.Limit_Filter_Positive_Distance,0,8)BTD(Port_Data.Data_Transfer[23],0,Q90R2KD.Write.Config.Limit_Filter_Negative_Distance,24,8)BTD(Port_Data.Data_Transfer[24],0,Q90R2KD.Write.Config.Limit_Filter_Negative_Distance,16,8)BTD(Port_Data.Data_Transfer[25],0,Q90R2KD.Write.Config.Limit_Filter_Negative_Distance,8,8)BTD(Port_Data.Data_Transfer[26],0,Q90R2KD.Write.Config.Limit_Filter_Negative_Distance,0,8)BTD(Port_Data.Data_Transfer[27],0,Q90R2KD.Write.Config.Primary_Output_Mode,0,8)BTD(Port_Data.Data_Transfer[28],0,Q90R2KD.Write.Config.Secondary_Output_Mode,0,8)OTU(Port_Data.Port_Read.[Port])OTL(Local_Control.6);
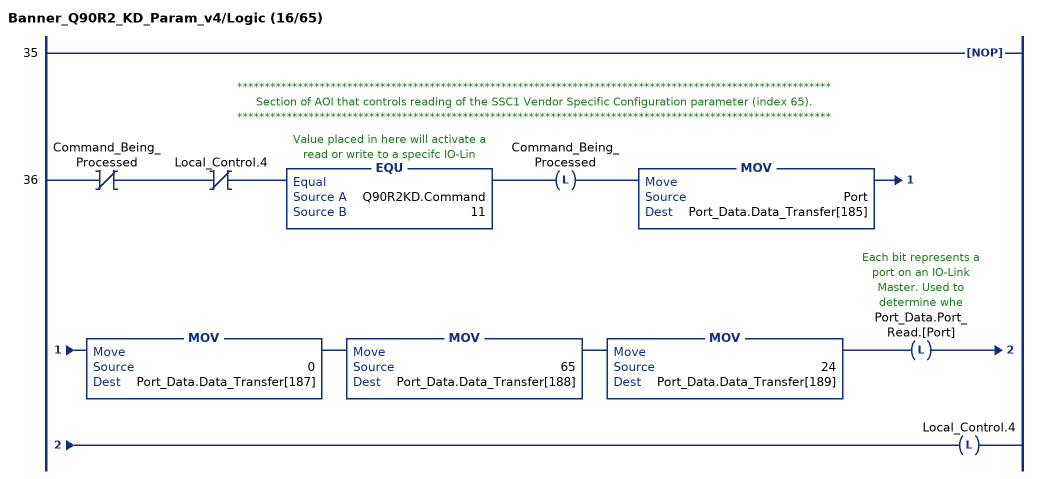
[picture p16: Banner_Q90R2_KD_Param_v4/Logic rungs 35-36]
   35: NOP();
   // ************************************************************************************************************
   // Section of AOI that controls reading of the SSC1 Vendor Specific Configuration parameter (index 65).
   // ************************************************************************************************************
   36: XIO(Command_Being_Processed)XIO(Local_Control.4)EQU(Q90R2KD.Command,11)OTL(Command_Being_Processed)MOV(Port,Port_Data.Data_Transfer[185])MOV(0,Port_Data.Data_Transfer[187])MOV(65,Port_Data.Data_Transfer[188])MOV(24,Port_Data.Data_Transfer[189])OTL(Port_Data.Port_Read.[Port])OTL(Local_Control.4);
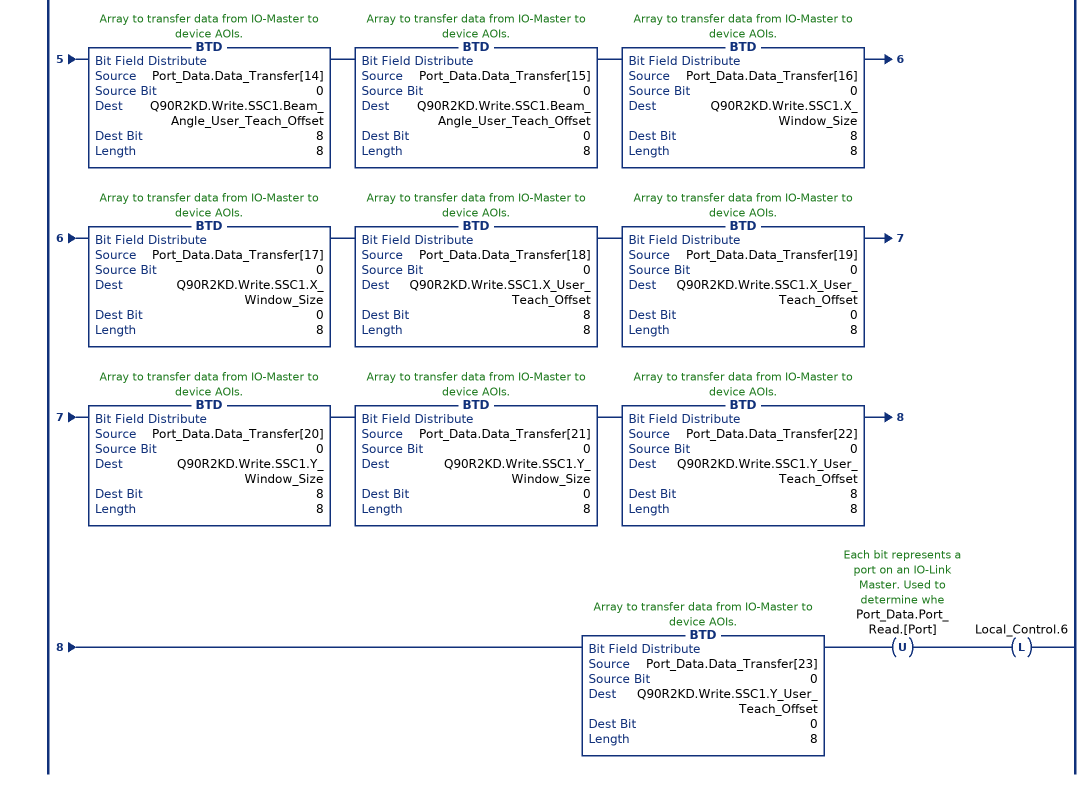
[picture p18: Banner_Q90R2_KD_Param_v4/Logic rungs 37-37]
   37: XIC(Local_Control.5)XIO(Local_Control.6)EQU(Q90R2KD.Command,11)BTD(Port_Data.Data_Transfer[0],0,Q90R2KD.Write.SSC1.Delay_On,24,8)BTD(Port_Data.Data_Transfer[1],0,Q90R2KD.Write.SSC1.Delay_On,16,8)BTD(Port_Data.Data_Transfer[2],0,Q90R2KD.Write.SSC1.Delay_On,8,8)BTD(Port_Data.Data_Transfer[3],0,Q90R2KD.Write.SSC1.Delay_On,0,8)BTD(Port_Data.Data_Transfer[4],0,Q90R2KD.Write.SSC1.Delay_Off,24,8)BTD(Port_Data.Data_Transfer[5],0,Q90R2KD.Write.SSC1.Delay_Off,16,8)BTD(Port_Data.Data_Transfer[6],0,Q90R2KD.Write.SSC1.Delay_Off,8,8)BTD(Port_Data.Data_Transfer[7],0,Q90R2KD.Write.SSC1.Delay_Off,0,8)BTD(Port_Data.Data_Transfer[8],0,Q90R2KD.Write.SSC1.Distance_Window_Size,8,8)BTD(Port_Data.Data_Transfer[9],0,Q90R2KD.Write.SSC1.Distance_Window_Size,0,8)BTD(Port_Data.Data_Transfer[10],0,Q90R2KD.Write.SSC1.Distance_User_Teach_Offset,8,8)BTD(Port_Data.Data_Transfer[11],0,Q90R2KD.Write.SSC1.Distance_User_Teach_Offset,0,8)BTD(Port_Data.Data_Transfer[12],0,Q90R2KD.Write.SSC1.Beam_Angle_Window_Size,8,8)BTD(Port_Data.Data_Transfer[13],0,Q90R2KD.Write.SSC1.Beam_Angle_Window_Size,0,8)BTD(Port_Data.Data_Transfer[14],0,Q90R2KD.Write.SSC1.Beam_Angle_User_Teach_Offset,8,8)BTD(Port_Data.Data_Transfer[15],0,Q90R2KD.Write.SSC1.Beam_Angle_User_Teach_Offset,0,8)BTD(Port_Data.Data_Transfer[16],0,Q90R2KD.Write.SSC1.X_Window_Size,8,8)BTD(Port_Data.Data_Transfer[17],0,Q90R2KD.Write.SSC1.X_Window_Size,0,8)BTD(Port_Data.Data_Transfer[18],0,Q90R2KD.Write.SSC1.X_User_Teach_Offset,8,8)BTD(Port_Data.Data_Transfer[19],0,Q90R2KD.Write.SSC1.X_User_Teach_Offset,0,8)BTD(Port_Data.Data_Transfer[20],0,Q90R2KD.Write.SSC1.Y_Window_Size,8,8)BTD(Port_Data.Data_Transfer[21],0,Q90R2KD.Write.SSC1.Y_Window_Size,0,8)BTD(Port_Data.Data_Transfer[22],0,Q90R2KD.Write.SSC1.Y_User_Teach_Offset,8,8)BTD(Port_Data.Data_Transfer[23],0,Q90R2KD.Write.SSC1.Y_User_Teach_Offset,0,8)OTU(Port_Data.Port_Read.[Port])OTL(Local_Control.6);
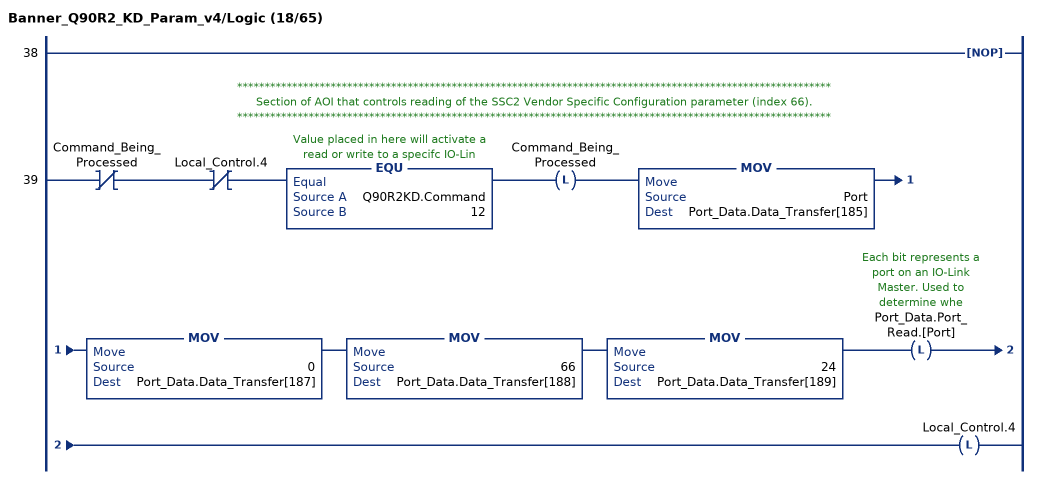
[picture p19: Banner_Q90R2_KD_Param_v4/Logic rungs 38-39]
   38: NOP();
   // ************************************************************************************************************
   // Section of AOI that controls reading of the SSC2 Vendor Specific Configuration parameter (index 66).
   // ************************************************************************************************************
   39: XIO(Command_Being_Processed)XIO(Local_Control.4)EQU(Q90R2KD.Command,12)OTL(Command_Being_Processed)MOV(Port,Port_Data.Data_Transfer[185])MOV(0,Port_Data.Data_Transfer[187])MOV(66,Port_Data.Data_Transfer[188])MOV(24,Port_Data.Data_Transfer[189])OTL(Port_Data.Port_Read.[Port])OTL(Local_Control.4);
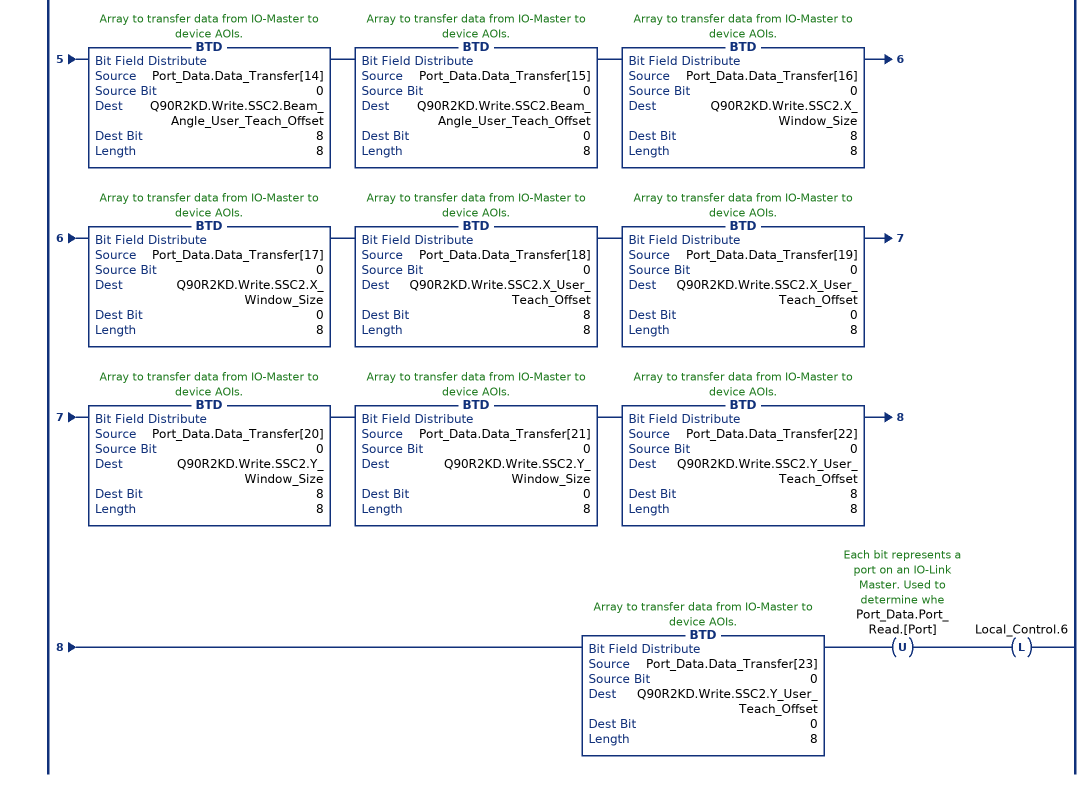
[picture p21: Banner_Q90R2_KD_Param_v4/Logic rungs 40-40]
   40: XIC(Local_Control.5)XIO(Local_Control.6)EQU(Q90R2KD.Command,12)BTD(Port_Data.Data_Transfer[0],0,Q90R2KD.Write.SSC2.Delay_On,24,8)BTD(Port_Data.Data_Transfer[1],0,Q90R2KD.Write.SSC2.Delay_On,16,8)BTD(Port_Data.Data_Transfer[2],0,Q90R2KD.Write.SSC2.Delay_On,8,8)BTD(Port_Data.Data_Transfer[3],0,Q90R2KD.Write.SSC2.Delay_On,0,8)BTD(Port_Data.Data_Transfer[4],0,Q90R2KD.Write.SSC2.Delay_Off,24,8)BTD(Port_Data.Data_Transfer[5],0,Q90R2KD.Write.SSC2.Delay_Off,16,8)BTD(Port_Data.Data_Transfer[6],0,Q90R2KD.Write.SSC2.Delay_Off,8,8)BTD(Port_Data.Data_Transfer[7],0,Q90R2KD.Write.SSC2.Delay_Off,0,8)BTD(Port_Data.Data_Transfer[8],0,Q90R2KD.Write.SSC2.Distance_Window_Size,8,8)BTD(Port_Data.Data_Transfer[9],0,Q90R2KD.Write.SSC2.Distance_Window_Size,0,8)BTD(Port_Data.Data_Transfer[10],0,Q90R2KD.Write.SSC2.Distance_User_Teach_Offset,8,8)BTD(Port_Data.Data_Transfer[11],0,Q90R2KD.Write.SSC2.Distance_User_Teach_Offset,0,8)BTD(Port_Data.Data_Transfer[12],0,Q90R2KD.Write.SSC2.Beam_Angle_Window_Size,8,8)BTD(Port_Data.Data_Transfer[13],0,Q90R2KD.Write.SSC2.Beam_Angle_Window_Size,0,8)BTD(Port_Data.Data_Transfer[14],0,Q90R2KD.Write.SSC2.Beam_Angle_User_Teach_Offset,8,8)BTD(Port_Data.Data_Transfer[15],0,Q90R2KD.Write.SSC2.Beam_Angle_User_Teach_Offset,0,8)BTD(Port_Data.Data_Transfer[16],0,Q90R2KD.Write.SSC2.X_Window_Size,8,8)BTD(Port_Data.Data_Transfer[17],0,Q90R2KD.Write.SSC2.X_Window_Size,0,8)BTD(Port_Data.Data_Transfer[18],0,Q90R2KD.Write.SSC2.X_User_Teach_Offset,8,8)BTD(Port_Data.Data_Transfer[19],0,Q90R2KD.Write.SSC2.X_User_Teach_Offset,0,8)BTD(Port_Data.Data_Transfer[20],0,Q90R2KD.Write.SSC2.Y_Window_Size,8,8)BTD(Port_Data.Data_Transfer[21],0,Q90R2KD.Write.SSC2.Y_Window_Size,0,8)BTD(Port_Data.Data_Transfer[22],0,Q90R2KD.Write.SSC2.Y_User_Teach_Offset,8,8)BTD(Port_Data.Data_Transfer[23],0,Q90R2KD.Write.SSC2.Y_User_Teach_Offset,0,8)OTU(Port_Data.Port_Read.[Port])OTL(Local_Control.6);
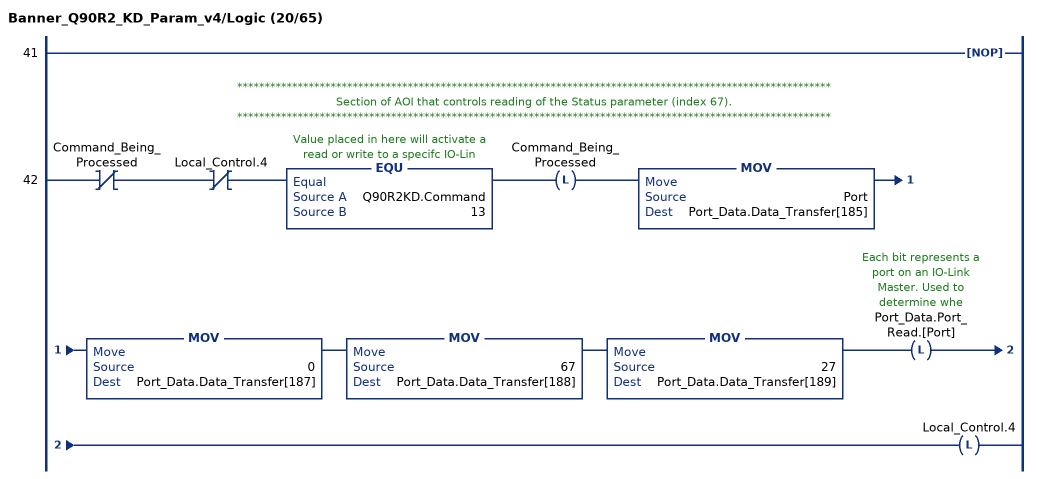
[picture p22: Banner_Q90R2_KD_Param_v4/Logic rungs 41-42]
   41: NOP();
   // ************************************************************************************************************
   // Section of AOI that controls reading of the Status parameter (index 67).
   // ************************************************************************************************************
   42: XIO(Command_Being_Processed)XIO(Local_Control.4)EQU(Q90R2KD.Command,13)OTL(Command_Being_Processed)MOV(Port,Port_Data.Data_Transfer[185])MOV(0,Port_Data.Data_Transfer[187])MOV(67,Port_Data.Data_Transfer[188])MOV(27,Port_Data.Data_Transfer[189])OTL(Port_Data.Port_Read.[Port])OTL(Local_Control.4);
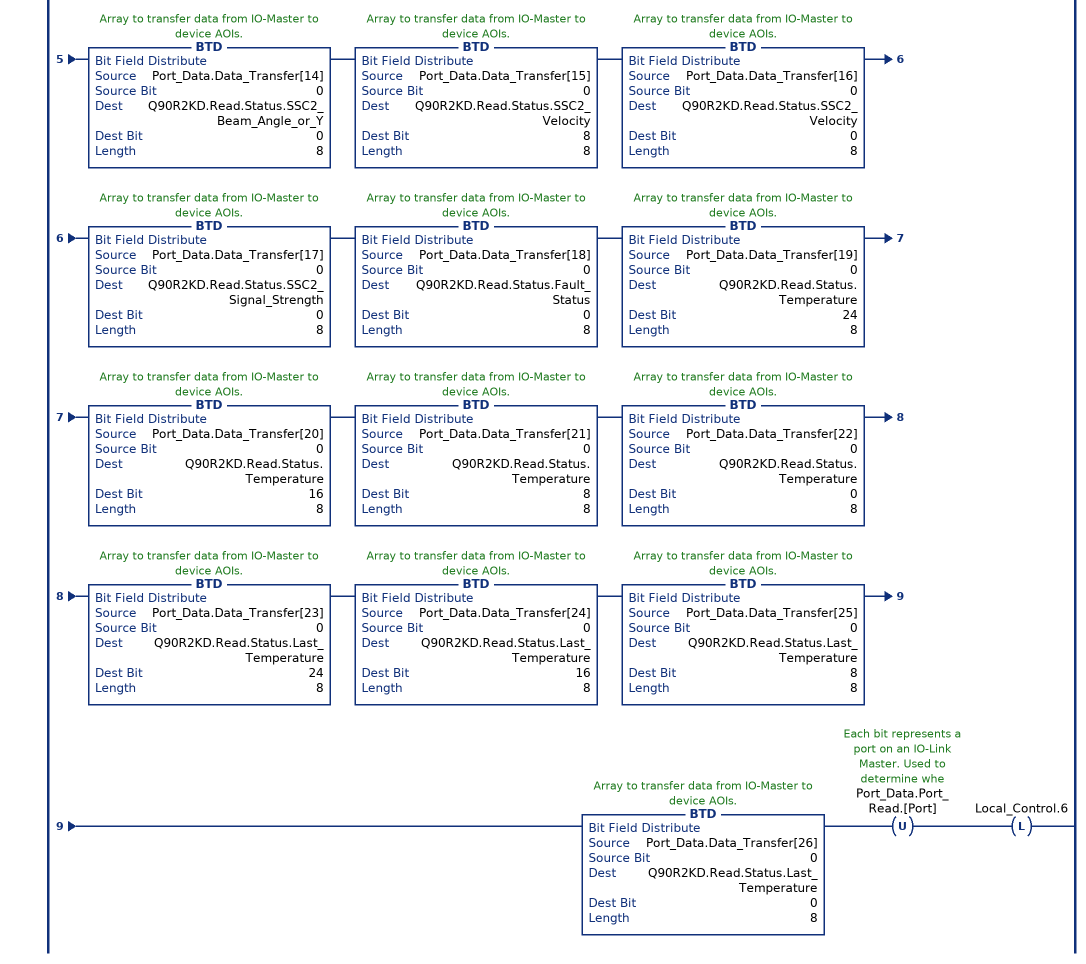
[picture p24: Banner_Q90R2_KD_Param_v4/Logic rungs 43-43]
   43: XIC(Local_Control.5)XIO(Local_Control.6)EQU(Q90R2KD.Command,13)BTD(Port_Data.Data_Transfer[0],0,Q90R2KD.Read.Status.SSC1_State,0,8)BTD(Port_Data.Data_Transfer[1],0,Q90R2KD.Read.Status.SSC1_Stability,0,8)BTD(Port_Data.Data_Transfer[2],0,Q90R2KD.Read.Status.SSC1_Distance_or_X,8,8)BTD(Port_Data.Data_Transfer[3],0,Q90R2KD.Read.Status.SSC1_Distance_or_X,0,8)BTD(Port_Data.Data_Transfer[4],0,Q90R2KD.Read.Status.SSC1_Beam_Angle_or_Y,8,8)BTD(Port_Data.Data_Transfer[5],0,Q90R2KD.Read.Status.SSC1_Beam_Angle_or_Y,0,8)BTD(Port_Data.Data_Transfer[6],0,Q90R2KD.Read.Status.SSC1_Velocity,8,8)BTD(Port_Data.Data_Transfer[7],0,Q90R2KD.Read.Status.SSC1_Velocity,0,8)BTD(Port_Data.Data_Transfer[8],0,Q90R2KD.Read.Status.SSC1_Signal_Strength,0,8)BTD(Port_Data.Data_Transfer[9],0,Q90R2KD.Read.Status.SSC2_State,0,8)BTD(Port_Data.Data_Transfer[10],0,Q90R2KD.Read.Status.SSC2_Stability,0,8)BTD(Port_Data.Data_Transfer[11],0,Q90R2KD.Read.Status.SSC2_Distance_or_X,8,8)BTD(Port_Data.Data_Transfer[12],0,Q90R2KD.Read.Status.SSC2_Distance_or_X,0,8)BTD(Port_Data.Data_Transfer[13],0,Q90R2KD.Read.Status.SSC2_Beam_Angle_or_Y,8,8)BTD(Port_Data.Data_Transfer[14],0,Q90R2KD.Read.Status.SSC2_Beam_Angle_or_Y,0,8)BTD(Port_Data.Data_Transfer[15],0,Q90R2KD.Read.Status.SSC2_Velocity,8,8)BTD(Port_Data.Data_Transfer[16],0,Q90R2KD.Read.Status.SSC2_Velocity,0,8)BTD(Port_Data.Data_Transfer[17],0,Q90R2KD.Read.Status.SSC2_Signal_Strength,0,8)BTD(Port_Data.Data_Transfer[18],0,Q90R2KD.Read.Status.Fault_Status,0,8)BTD(Port_Data.Data_Transfer[19],0,Q90R2KD.Read.Status.Temperature,24,8)BTD(Port_Data.Data_Transfer[20],0,Q90R2KD.Read.Status.Temperature,16,8)BTD(Port_Data.Data_Transfer[21],0,Q90R2KD.Read.Status.Temperature,8,8)BTD(Port_Data.Data_Transfer[22],0,Q90R2KD.Read.Status.Temperature,0,8)BTD(Port_Data.Data_Transfer[23],0,Q90R2KD.Read.Status.Last_Temperature,24,8)BTD(Port_Data.Data_Transfer[24],0,Q90R2KD.Read.Status.Last_Temperature,16,8)BTD(Port_Data.Data_Transfer[25],0,Q90R2KD.Read.Status.Last_Temperature,8,8)BTD(Port_Data.Data_Transfer[26],0,Q90R2KD.Read.Status.Last_Temperature,0,8)OTU(Port_Data.Port_Read.[Port])OTL(Local_Control.6);
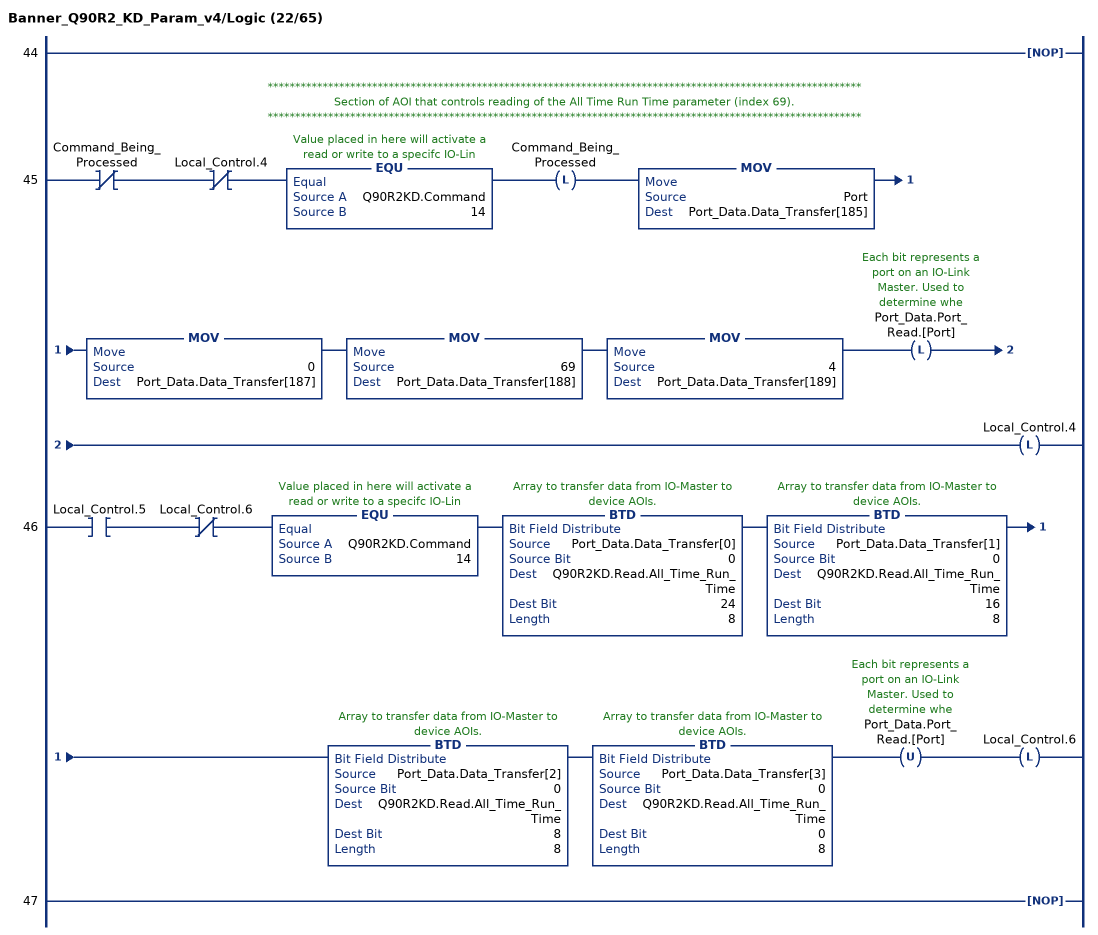
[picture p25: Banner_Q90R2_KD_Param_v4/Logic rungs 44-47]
   44: NOP();
   // ************************************************************************************************************
   // Section of AOI that controls reading of the All Time Run Time parameter (index 69).
   // ************************************************************************************************************
   45: XIO(Command_Being_Processed)XIO(Local_Control.4)EQU(Q90R2KD.Command,14)OTL(Command_Being_Processed)MOV(Port,Port_Data.Data_Transfer[185])MOV(0,Port_Data.Data_Transfer[187])MOV(69,Port_Data.Data_Transfer[188])MOV(4,Port_Data.Data_Transfer[189])OTL(Port_Data.Port_Read.[Port])OTL(Local_Control.4);
   46: XIC(Local_Control.5)XIO(Local_Control.6)EQU(Q90R2KD.Command,14)BTD(Port_Data.Data_Transfer[0],0,Q90R2KD.Read.All_Time_Run_Time,24,8)BTD(Port_Data.Data_Transfer[1],0,Q90R2KD.Read.All_Time_Run_Time,16,8)BTD(Port_Data.Data_Transfer[2],0,Q90R2KD.Read.All_Time_Run_Time,8,8)BTD(Port_Data.Data_Transfer[3],0,Q90R2KD.Read.All_Time_Run_Time,0,8)OTU(Port_Data.Port_Read.[Port])OTL(Local_Control.6);
   47: NOP();
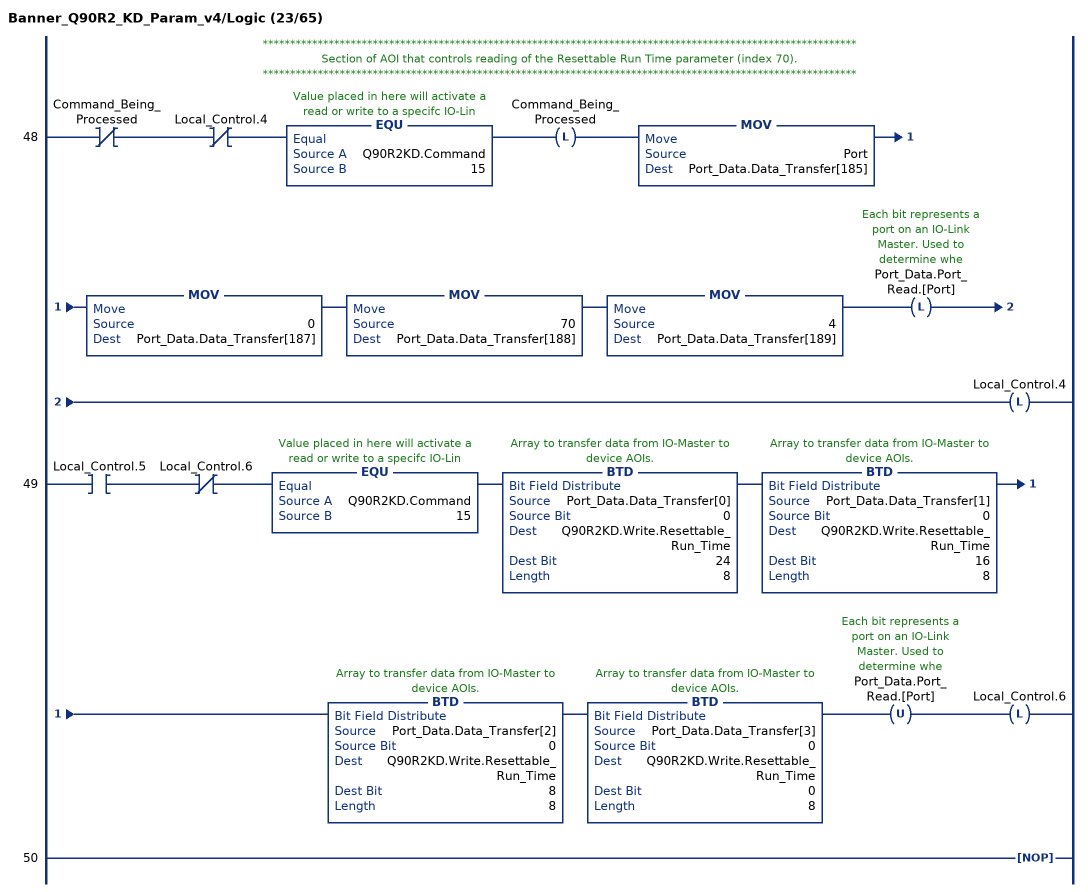
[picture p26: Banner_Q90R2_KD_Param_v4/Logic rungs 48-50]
   // ************************************************************************************************************
   // Section of AOI that controls reading of the Resettable Run Time parameter (index 70).
   // ************************************************************************************************************
   48: XIO(Command_Being_Processed)XIO(Local_Control.4)EQU(Q90R2KD.Command,15)OTL(Command_Being_Processed)MOV(Port,Port_Data.Data_Transfer[185])MOV(0,Port_Data.Data_Transfer[187])MOV(70,Port_Data.Data_Transfer[188])MOV(4,Port_Data.Data_Transfer[189])OTL(Port_Data.Port_Read.[Port])OTL(Local_Control.4);
   49: XIC(Local_Control.5)XIO(Local_Control.6)EQU(Q90R2KD.Command,15)BTD(Port_Data.Data_Transfer[0],0,Q90R2KD.Write.Resettable_Run_Time,24,8)BTD(Port_Data.Data_Transfer[1],0,Q90R2KD.Write.Resettable_Run_Time,16,8)BTD(Port_Data.Data_Transfer[2],0,Q90R2KD.Write.Resettable_Run_Time,8,8)BTD(Port_Data.Data_Transfer[3],0,Q90R2KD.Write.Resettable_Run_Time,0,8)OTU(Port_Data.Port_Read.[Port])OTL(Local_Control.6);
   50: NOP();
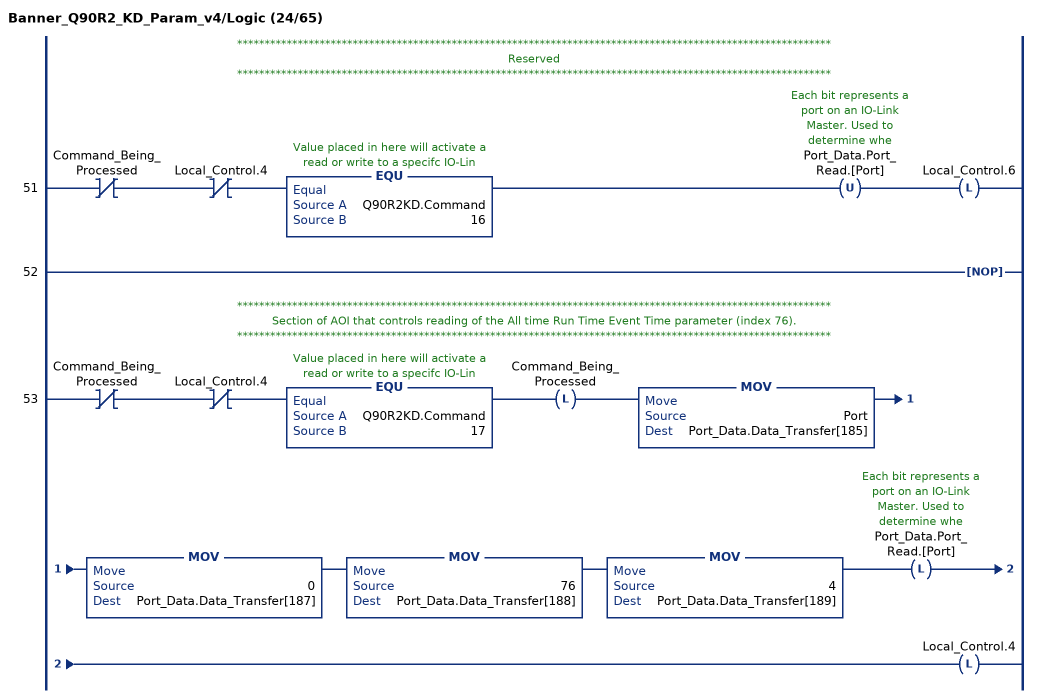
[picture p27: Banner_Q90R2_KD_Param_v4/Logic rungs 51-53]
   // ************************************************************************************************************
   // Reserved
   // ************************************************************************************************************
   51: XIO(Command_Being_Processed)XIO(Local_Control.4)EQU(Q90R2KD.Command,16)OTU(Port_Data.Port_Read.[Port])OTL(Local_Control.6);
   52: NOP();
   // ************************************************************************************************************
   // Section of AOI that controls reading of the All time Run Time Event Time parameter (index 76).
   // ************************************************************************************************************
   53: XIO(Command_Being_Processed)XIO(Local_Control.4)EQU(Q90R2KD.Command,17)OTL(Command_Being_Processed)MOV(Port,Port_Data.Data_Transfer[185])MOV(0,Port_Data.Data_Transfer[187])MOV(76,Port_Data.Data_Transfer[188])MOV(4,Port_Data.Data_Transfer[189])OTL(Port_Data.Port_Read.[Port])OTL(Local_Control.4);
